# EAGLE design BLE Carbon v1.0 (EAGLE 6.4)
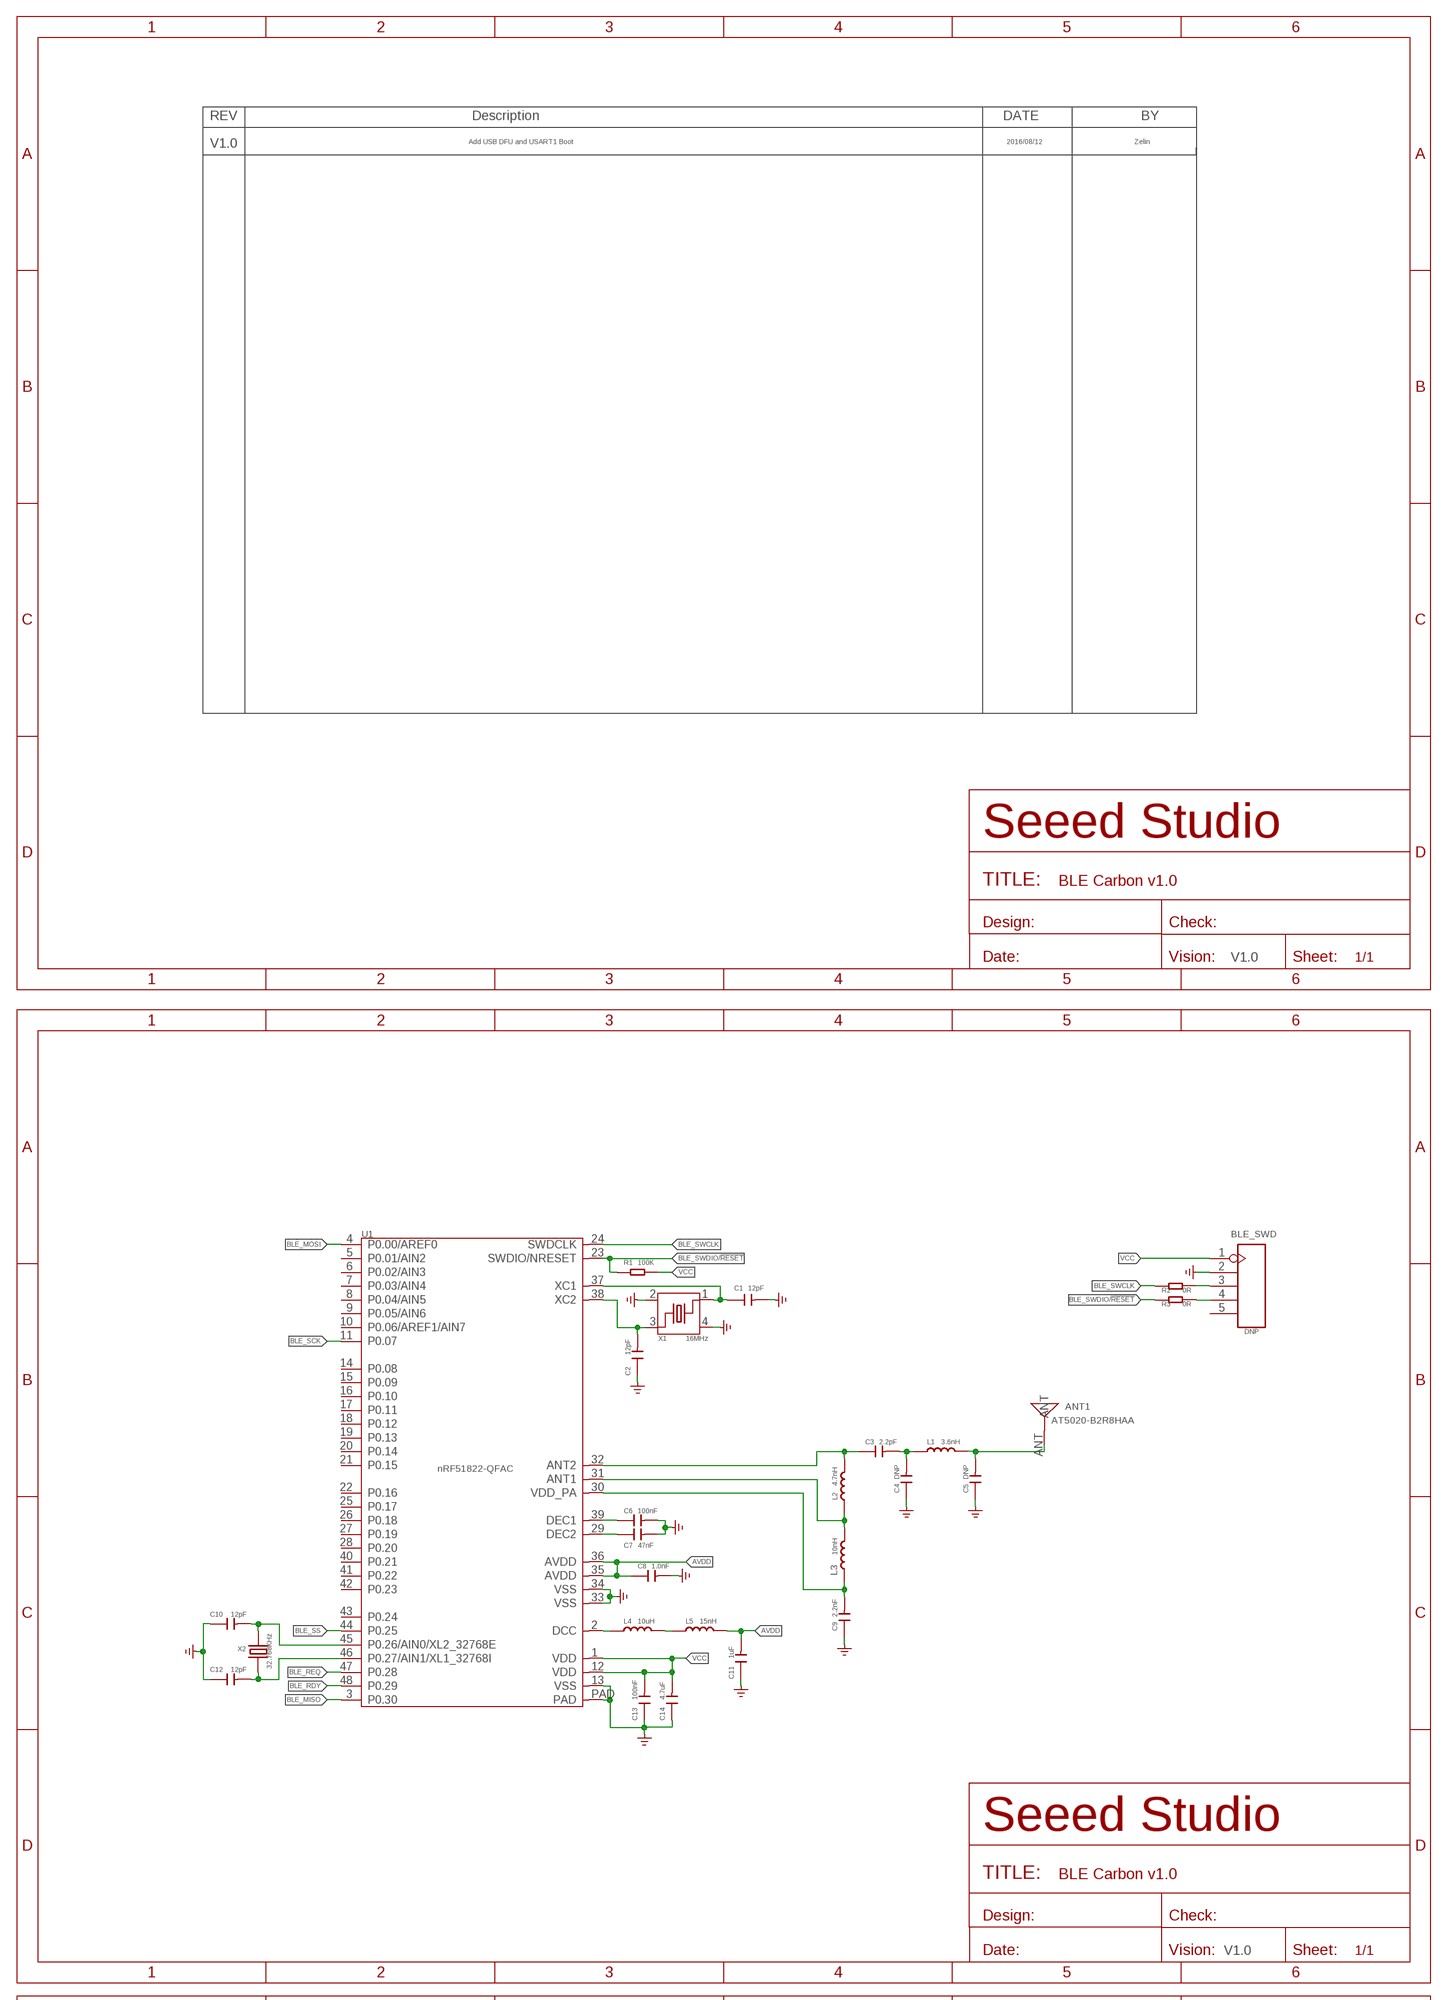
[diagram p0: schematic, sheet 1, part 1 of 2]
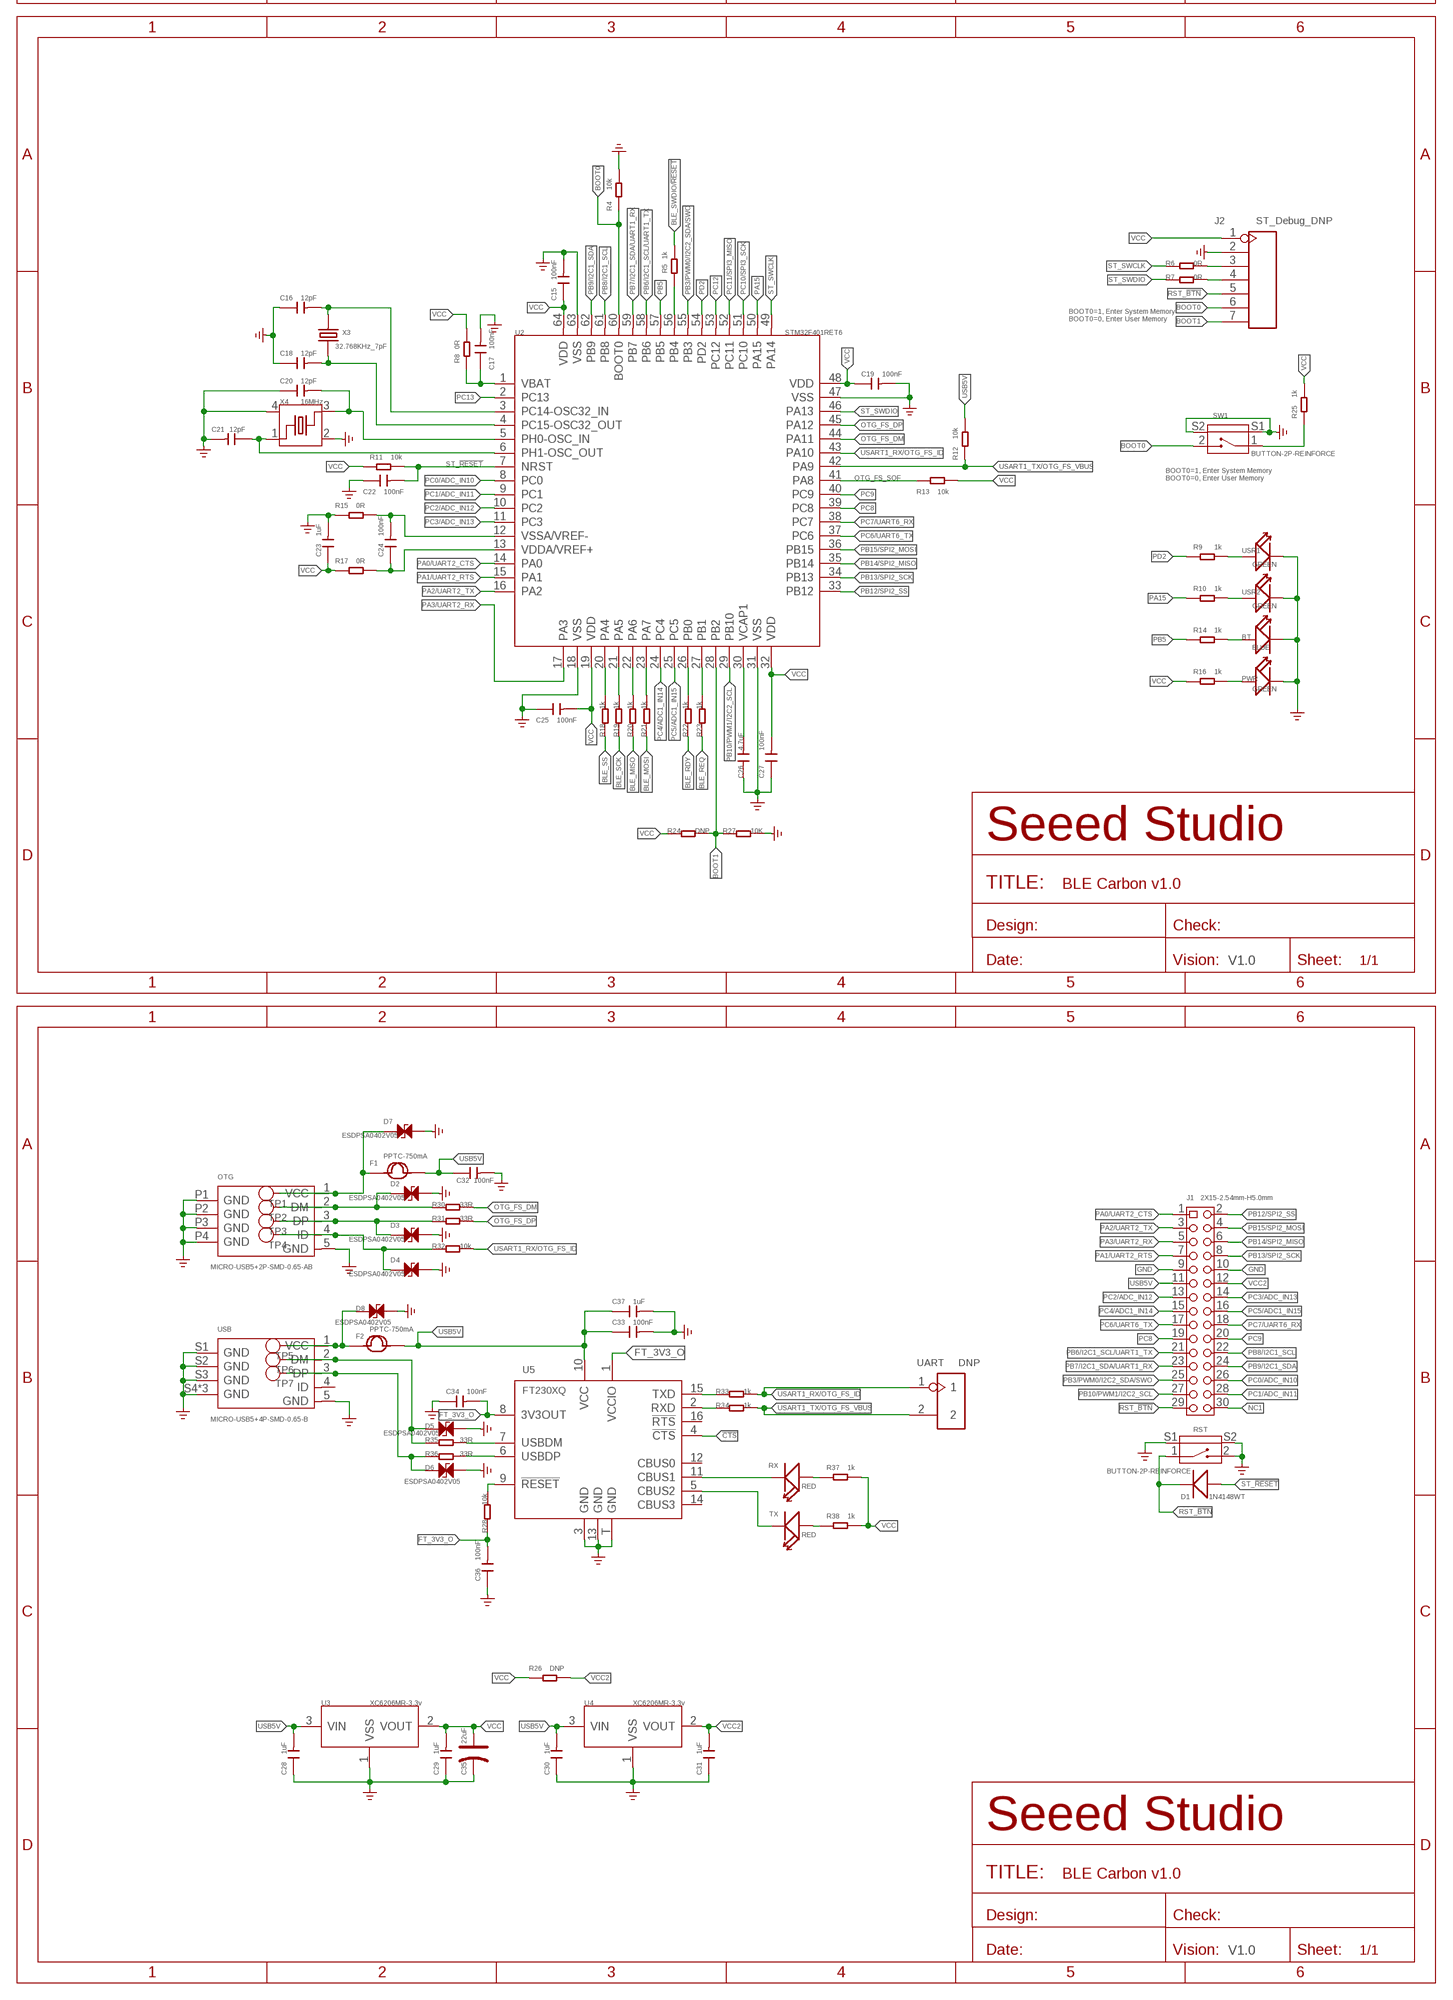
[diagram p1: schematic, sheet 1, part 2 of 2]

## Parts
ANT1  AT5020-B2R8HAA  ANTENNA-AN2051-2.4G  [ANT-SMD2P-5.05X2X1.07MM]
BLE_SWD  DNP  HEADER-5P-2.54  [H5-2.54]
BT  BLUE  LED'0402'  [LED-0402]
C1  12pF  C-0402  [C0402]
C2  12pF  C-0402  [C0402]
C3  2.2pF  C-0402  [C0402]
C4  DNP  C-0402  [C0402]
C5  DNP  C-0402  [C0402]
C6  100nF  C-0402  [C0402]
C7  47nF  C-0402  [C0402]
C8  1.0nF  C-0402  [C0402]
C9  2.2nF  C-0402  [C0402]
C10  12pF  C-0402  [C0402]
C11  1uF  C-0402  [C0402]
C12  12pF  C-0402  [C0402]
C13  100nF  C-0402  [C0402]
C14  4.7uF  C-0603  [C0603]
C15  100nF  C-0402  [C0402]
C16  12pF  C-0402  [C0402]
C17  100nF  C-0402  [C0402]
C18  12pF  C-0402  [C0402]
C19  100nF  C-0402  [C0402]
C20  12pF  C-0402  [C0402]
C21  12pF  C-0402  [C0402]
C22  100nF  C-0402  [C0402]
C23  1uF  C-0402  [C0402]
C24  100nF  C-0402  [C0402]
C25  100nF  C-0402  [C0402]
C26  4.7uF  C-0603  [C0603]
C27  100nF  C-0402  [C0402]
C28  1uF  C-0603  [C0603]
C29  1uF  C-0603  [C0603]
C30  1uF  C-0603  [C0603]
C31  1uF  C-0603  [C0603]
C32  100nF  C-0402  [C0402]
C33  100nF  C-0402  [C0402]
C34  100nF  C-0402  [C0402]
C35  22uF  CAP-AVX-A  [AVX-A]
C36  100nF  C-0402  [C0402]
C37  1uF  C-0603  [C0603]
D1  1N4148WT  D'0603'  [SOD523]
D2  ESDPSA0402V05  D-ESD-2P-DOUBLE  [ESD-0402]
D3  ESDPSA0402V05  D-ESD-2P-DOUBLE  [ESD-0402]
D4  ESDPSA0402V05  D-ESD-2P-DOUBLE  [ESD-0402]
D5  ESDPSA0402V05  D-ESD-2P-DOUBLE  [ESD-0402]
D6  ESDPSA0402V05  D-ESD-2P-DOUBLE  [ESD-0402]
D7  ESDPSA0402V05  D-ESD-2P-DOUBLE  [ESD-0402]
D8  ESDPSA0402V05  D-ESD-2P-DOUBLE  [ESD-0402]
F1  PPTC-750mA  FUSE'1206'  [F1206]
F2  PPTC-750mA  FUSE'1206'  [F1206]
J1  2X15-2.54mm-H5.0mm  HEADER-2X15P-2.54  [H2X15-2.54]
J2  ST_Debug_DNP  HEADER-7P  [H7-2.54]
L1  3.6nH  L'0402'  [L0402]
L2  4.7nH  L'0402'  [L0402]
L3  10nH  L'0402'  [L0402]
L4  10uH  L'0603'  [L0603]
L5  15nH  L'0402'  [L0402]
OTG  MICRO-USB5+2P-SMD-0.65-AB  MICRO-USB5+4P'ALX-MC-5F-036'  [MICRO-USB5+2P-SMD-0.65-AB]
PWR  GREEN  LED'0402'  [LED-0402]
R1  100K  R-0402  [R0402]
R2  0R  R-0402  [R0402]
R3  0R  R-0402  [R0402]
R4  10k  R-0402  [R0402]
R5  1k  R-0402  [R0402]
R6  0R  R-0402  [R0402]
R7  0R  R-0402  [R0402]
R8  0R  R-0402  [R0402]
R9  1k  R-0402  [R0402]
R10  1k  R-0402  [R0402]
R11  10k  R-0402  [R0402]
R12  10k  R-0402  [R0402]
R13  10k  R-0402  [R0402]
R14  1k  R-0402  [R0402]
R15  0R  R-0402  [R0402]
R16  1k  R-0402  [R0402]
R17  0R  R-0402  [R0402]
R18  1k  R-0402  [R0402]
R19  1k  R-0402  [R0402]
R20  1k  R-0402  [R0402]
R21  1k  R-0402  [R0402]
R22  1k  R-0402  [R0402]
R23  1k  R-0402  [R0402]
R24  DNP  R-0402  [R0402]
R25  1k  R-0402  [R0402]
R26  DNP  R-0402  [R0402]
R27  10K  R-0402  [R0402]
R28  10k  R-0402  [R0402]
R30  33R  R-0402  [R0402]
R31  33R  R-0402  [R0402]
R32  10k  R-0402  [R0402]
R33  1k  R-0402  [R0402]
R34  1k  R-0402  [R0402]
R35  33R  R-0402  [R0402]
R36  33R  R-0402  [R0402]
R37  1k  R-0402  [R0402]
R38  1k  R-0402  [R0402]
RST  BUTTON-2P-REINFORCE  [4P-SMD-4.7X3.5X1.8]
RX  RED  LED'0402'  [LED-0402]
SW1  BUTTON-2P-REINFORCE  [4P-SMD-4.7X3.5X1.8]
TP1  VBUS  TEST-POINT'4545'  [TP-D45MIL]
TP2  DM  TEST-POINT'4545'  [TP-D45MIL]
TP3  DP  TEST-POINT'4545'  [TP-D45MIL]
TP4  ID  TEST-POINT'4545'  [TP-D45MIL]
TP5  VBUS  TEST-POINT'4545'  [TP-D45MIL]
TP6  DM  TEST-POINT'4545'  [TP-D45MIL]
TP7  DP  TEST-POINT'4545'  [TP-D45MIL]
TX  RED  LED'0402'  [LED-0402]
U1  nRF51822-QFAC  NRF51822QFAA  [QFN48-6X6MM]
U2  STM32F401RET6  MCU-STM32F401XD/XE  [LQFP64-0.5-10X10MM]
U3  XC6206MR-3.3v  XC6206MR  [SOT23]
U4  XC6206MR-3.3v  XC6206MR  [SOT23]
U5  FT230XQ  FT230X  [QFN16]
UART  DNP  HEADER-2P-65/35MIL  [H2-2.54]
USB  MICRO-USB5+4P-SMD-0.65-B  MICRO-USB5+4P'5+4P'  [MICRO-USB5+4P-SMD-0.65-B]
USR1  GREEN  LED'0402'  [LED-0402]
USR2  GREEN  LED'0402'  [LED-0402]
X1  16MHz  CRYSTAL-4P  [X4-SMD-3.2X2.5X0.7MM]
X2  32.768KHz  CRYSTAL-3215  [2P-SMD-3.2X1.5]
X3  32.768KHz_7pF  CRYSTAL-3215  [2P-SMD-3.2X1.5]
X4  16MHz  CRYSTAL-4P  [X4-SMD-3.2X2.5X0.7MM]

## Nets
!CTS: U5.4(!CTS)
ANT1: L2.1 L3.2 U1.31(ANT1)
ANT2: C3.1 L2.2 U1.32(ANT2)
AVDD: C8.1 C11.2 L5.2 U1.35(AVDD) U1.36(AVDD)
BLE_MISO: R20.1 U1.3(P0.30)
BLE_MOSI: R21.1 U1.4(P0.00/AREF0)
BLE_RDY: R22.1 U1.48(P0.29)
BLE_REQ: R23.1 U1.47(P0.28)
BLE_SCK: R19.1 U1.11(P0.07)
BLE_SS: R18.1 U1.44(P0.25)
BLE_SWCLK: R2.1 U1.24(SWDCLK)
BLE_SWDIO/!RESET: R1.1 R3.1 R5.2 U1.23(SWDIO/NRESET)
BOOT0: J2.6 R4.1 SW1.2 U2.60(BOOT0)
BOOT1: J2.7 R24.2 R27.1 U2.28(PB2)
FT_3V3_O: C34.2 C36.2 R28.1 U5.1(VCCIO) U5.8(3V3OUT)
GND: BLE_SWD.2 BT.- C1.2 C2.1 C4.1 C5.1 C6.2 C7.2 C8.2 C9.1 C10.1 C11.1 C12.1 C13.1 C14.1 C15.2 C16.1 C17.2 C18.1 C19.2 C20.1 C21.2 C22.1 C23.2 C25.1 C26.1 C27.1 C28.1 C29.1 C30.1 C31.1 C32.2 C33.2 C34.1 C35.- C36.1 C37.2 D2.2 D3.2 D4.2 D5.2 D6.2 D7.2 D8.2 J1.9 J1.10 J2.2 OTG.5(GND) OTG.P1(GND) OTG.P2(GND) OTG.P3(GND) OTG.P4(GND) PWR.- R4.2 R15.1 R27.2 RST.2 RST.S1 RST.S2 SW1.S1 SW1.S2 U1.13(VSS) U1.33(VSS) U1.34(VSS) U1.PAD U2.18(VSS) U2.31(VSS) U2.47(VSS) U2.63(VSS) U3.1(VSS) U4.1(VSS) U5.3(GND) U5.13(GND) U5.T(GND) USB.5(GND) USB.S1(GND) USB.S2(GND) USB.S3(GND) USB.S4(GND) USB.S5(GND) USB.S6(GND) USR1.- USR2.- X1.2 X1.4 X4.2 X4.4 ; supply symbol labelled GND_POWER
N$1: ANT1.ANT C5.2 L1.2
N$2: C2.2 U1.38(XC2) X1.3
N$3: C7.1 U1.29(DEC2)
N$4: C6.1 U1.39(DEC1)
N$5: C1.1 U1.37(XC1) X1.1
N$6: L4.1 U1.2(DCC)
N$7: L4.2 L5.1
N$8: C3.2 C4.2 L1.1
N$9: C26.2 U2.30(VCAP1)
N$10: J2.3 R6.2
N$11: D4.1 OTG.4(ID) R32.1 TP4.T
N$12: C21.1 U2.6(PH1-OSC_OUT) X4.1
N$13: C20.2 U2.5(PH0-OSC_IN) X4.3
N$14: D2.1 OTG.2(DM) R30.1 TP2.T
N$15: D3.1 OTG.3(DP) R31.1 TP3.T
N$17: D8.1 F2.1 TP5.T USB.1(VCC)
N$18: C17.1 R8.1 U2.1(VBAT)
N$19: R18.2 U2.20(PA4)
N$20: R19.2 U2.21(PA5)
N$21: R20.2 U2.22(PA6)
N$22: R21.2 U2.23(PA7)
N$23: R22.2 U2.26(PB0)
N$24: R23.2 U2.27(PB1)
N$25: R25.1 SW1.1
N$26: C24.2 R15.2 U2.12(VSSA/VREF-)
N$27: C24.1 R17.2 U2.13(VDDA/VREF+)
N$28: BLE_SWD.4 R3.2
N$29: J2.4 R7.2
N$30: R35.2 U5.7(USBDM)
N$31: R9.2 USR1.+
N$32: R36.2 U5.6(USBDP)
N$33: R33.1 U5.15(TXD)
N$34: R34.1 U5.2(RXD)
N$35: R10.2 USR2.+
N$36: BT.+ R14.2
N$37: R5.1 U2.56(PB4)
N$38: R28.2 U5.9(!RESET)
N$39: D7.1 F1.1 OTG.1(VCC) TP1.T
N$40: BLE_SWD.3 R2.2
N$41: RX.- U5.11(CBUS1)
N$42: PWR.+ R16.2
N$43: TX.- U5.5(CBUS2)
N$44: R37.1 RX.+
N$45: R38.1 TX.+
N$46: D5.1 R35.1 TP6.T USB.2(DM)
N$47: D6.1 R36.1 TP7.T USB.3(DP)
NC1: J1.30
OTG_FS_DM: R30.2 U2.44(PA11)
OTG_FS_DP: R31.2 U2.45(PA12)
OTG_FS_SOF: R13.1 U2.41(PA8)
PA0/UART2_CTS: J1.1 U2.14(PA0)
PA1/UART2_RTS: J1.7 U2.15(PA1)
PA2/UART2_TX: J1.3 U2.16(PA2)
PA3/UART2_RX: J1.5 U2.17(PA3)
PA15: R10.1 U2.50(PA15)
PB3/PWM0/I2C2_SDA/SWO: J1.25 U2.55(PB3)
PB5: R14.1 U2.57(PB5)
PB6/I2C1_SCL/UART1_TX: J1.21 U2.58(PB6)
PB7/I2C1_SDA/UART1_RX: J1.23 U2.59(PB7)
PB8/I2C1_SCL: J1.22 U2.61(PB8)
PB9/I2C1_SDA: J1.24 U2.62(PB9)
PB10/PWM1/I2C2_SCL: J1.27 U2.29(PB10)
PB12/SPI2_SS: J1.2 U2.33(PB12)
PB13/SPI2_SCK: J1.8 U2.34(PB13)
PB14/SPI2_MISO: J1.6 U2.35(PB14)
PB15/SPI2_MOSI: J1.4 U2.36(PB15)
PC0/ADC_IN10: J1.26 U2.8(PC0)
PC1/ADC_IN11: J1.28 U2.9(PC1)
PC2/ADC_IN12: J1.13 U2.10(PC2)
PC3/ADC_IN13: J1.14 U2.11(PC3)
PC4/ADC1_IN14: J1.15 U2.24(PC4)
PC5/ADC1_IN15: J1.16 U2.25(PC5)
PC6/UART6_TX: J1.17 U2.37(PC6)
PC7/UART6_RX: J1.18 U2.38(PC7)
PC8: J1.19 U2.39(PC8)
PC9: J1.20 U2.40(PC9)
PC10/SPI3_SCK: U2.51(PC10)
PC11/SPI3_MISO: U2.52(PC11)
PC12: U2.53(PC12)
PC13: U2.2(PC13)
PD2: R9.1 U2.54(PD2)
RST_!BTN: D1.- J1.29 J2.5 RST.1
ST_!RESET: C22.2 D1.+ R11.2 U2.7(NRST)
ST_SWCLK: R6.1 U2.49(PA14)
ST_SWDIO: R7.1 U2.46(PA13)
USART1_RX/OTG_FS_ID: R32.2 R33.2 U2.43(PA10) UART.1
USART1_TX/OTG_FS_VBUS: R12.1 R34.2 U2.42(PA9) UART.2
USB5V: C28.2 C30.2 C32.1 C33.1 C37.1 F1.2 F2.2 J1.11 R12.2 U3.3(VIN) U4.3(VIN) U5.10(VCC)
VCC: BLE_SWD.1 C13.2 C14.2 C15.1 C19.1 C23.1 C25.2 C27.2 C29.2 C35.+ J2.1 R1.2 R8.2 R11.1 R13.2 R16.1 R17.1 R24.1 R25.2 R26.1 R37.2 R38.2 U1.1(VDD) U1.12(VDD) U2.19(VDD) U2.32(VDD) U2.48(VDD) U2.64(VDD) U3.2(VOUT)
VCC2: C31.2 J1.12 R26.2 U4.2(VOUT)
VDD_PA: C9.2 L3.1 U1.30(VDD_PA)
XL1_32768I: C12.2 U1.46(P0.27/AIN1/XL1_32768I) X2.1
XL1_32768I1: C18.2 U2.4(PC15-OSC32_OUT) X3.1
XL2_32768E: C10.2 U1.45(P0.26/AIN0/XL2_32768E) X2.2
XL2_32768E1: C16.2 U2.3(PC14-OSC32_IN) X3.2
Unconnected: BLE_SWD.5 U1.5(P0.01/AIN2) U1.6(P0.02/AIN3) U1.7(P0.03/AIN4) U1.8(P0.04/AIN5) U1.9(P0.05/AIN6) U1.10(P0.06/AREF1/AIN7) U1.14(P0.08) U1.15(P0.09) U1.16(P0.10) U1.17(P0.11) U1.18(P0.12) U1.19(P0.13) U1.20(P0.14) U1.21(P0.15) U1.22(P0.16) U1.25(P0.17) U1.26(P0.18) U1.27(P0.19) U1.28(P0.20) U1.40(P0.21) U1.41(P0.22) U1.42(P0.23) U1.43(P0.24) U5.12(CBUS0) U5.14(CBUS3) U5.16(!RTS) USB.4(ID)

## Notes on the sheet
- Add USB DFU and USART1 Boot | 2016/08/12 | Zelin
- V1.0
- V1.0
- V1.0
- BOOT0=1, Enter System Memory
  BOOT0=0, Enter User Memory
- BOOT0=1, Enter System Memory
  BOOT0=0, Enter User Memory
- V1.0
- V1.0

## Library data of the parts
ANT1 = Connector-new:ANTENNA-AN2051-2.4G: Multilayer Chip Antenna for 2.4GHz Wireless Communication
BLE_SWD = Connector-update:HEADER-5P
BT PWR RX TX USR1 USR2 = Discrete:LED*
C1-C34 C36 C37 = Discrete:C*: Ceramic Capacitors
C35 = Discrete:CAP*: Electrolytic Capacitors,Tantalum Capacitors and Super Capacitors
D1 = Discrete:D*
D2-D8 = Discrete-new:D-ESD-2P-DOUBLE
F1 F2 = Discrete:FUSE
J1 = Connector-update:HEADER-2X15P
J2 = Connector-new:HEADER-7P
L1-L5 = Discrete:L*
OTG = Connector-new:MICRO-USB5+4P: 5+4P-SMD-0.65-B:320010000;5+2P-SMD-0.65-AB:340032001; MPN: ALX-MC-5F-036; SKU: 320010025
R1-R28 R30-R38 = Discrete:R*
RST SW1 = Discrete:BUTTON-2P-REINFORCE: TS-1188E http://www.best-dz.com/?thread-374-2.html SMD Button
TP1-TP7 = Discrete-new:TEST-POINT; PARTNO: DNP
U1 = AMLib_New:NRF51822QFAA: Multi-protocol Blutooth 4.0 low energy /2. GHz RF SoC
U2 = AMLib_U2N:MCU-STM32F401XD/XE
U3 U4 = IC:XC6206: LOW ESR Cap.Compatible Positive Voltage Regulators
U5 = AMLib_New:FT230X
UART = Connector-update:HEADER-2P
USB = Connector-new:MICRO-USB5+4P: 5+4P-SMD-0.65-B:320010000;5+2P-SMD-0.65-AB:340032001
X1 X4 = Discrete-new:CRYSTAL-4P
X2 X3 = Discrete:CRYSTAL*: CRYSTAL

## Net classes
0 default: width 0.152 mm, drill 0.254 mm, clearance 0.152 mm
1 vcc: width 0.203 mm

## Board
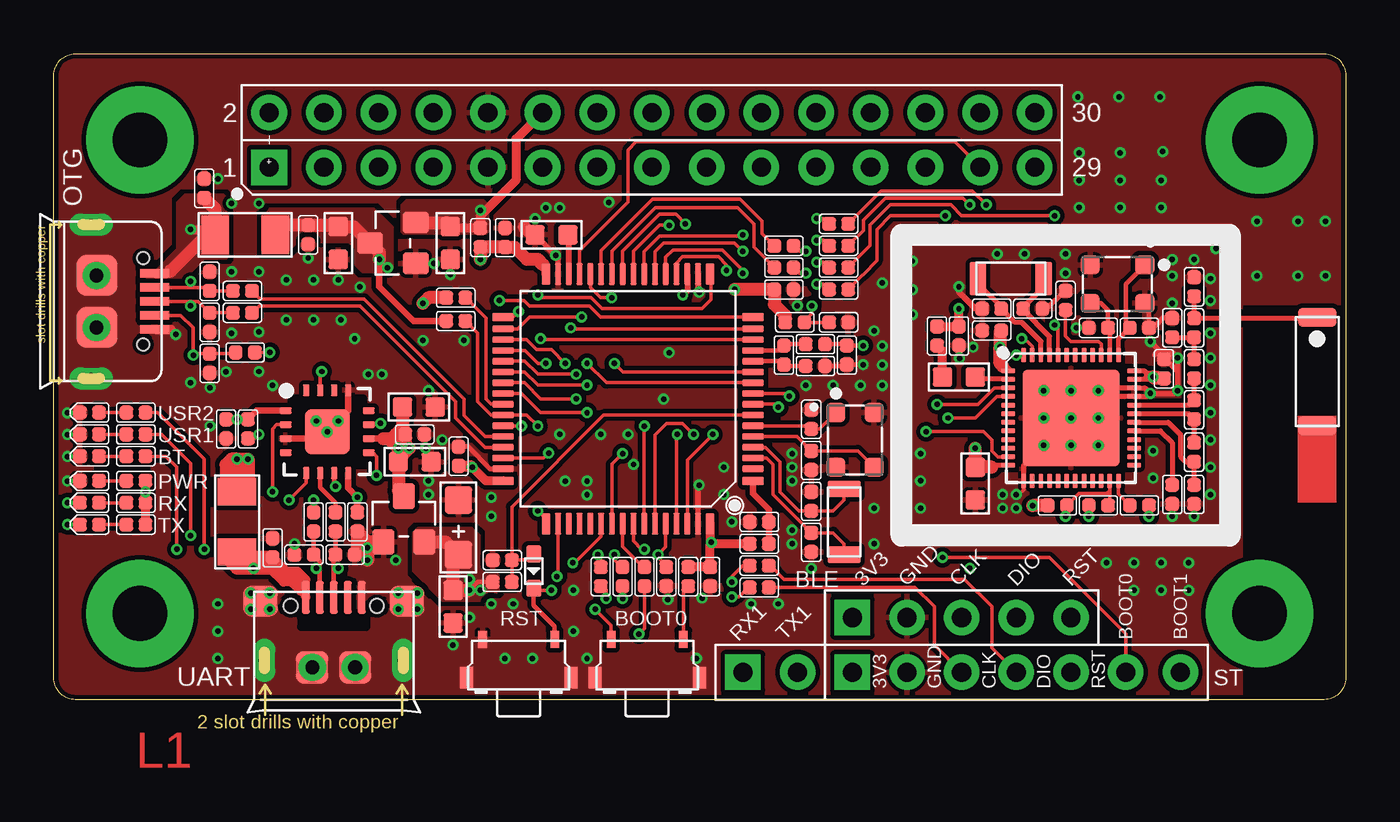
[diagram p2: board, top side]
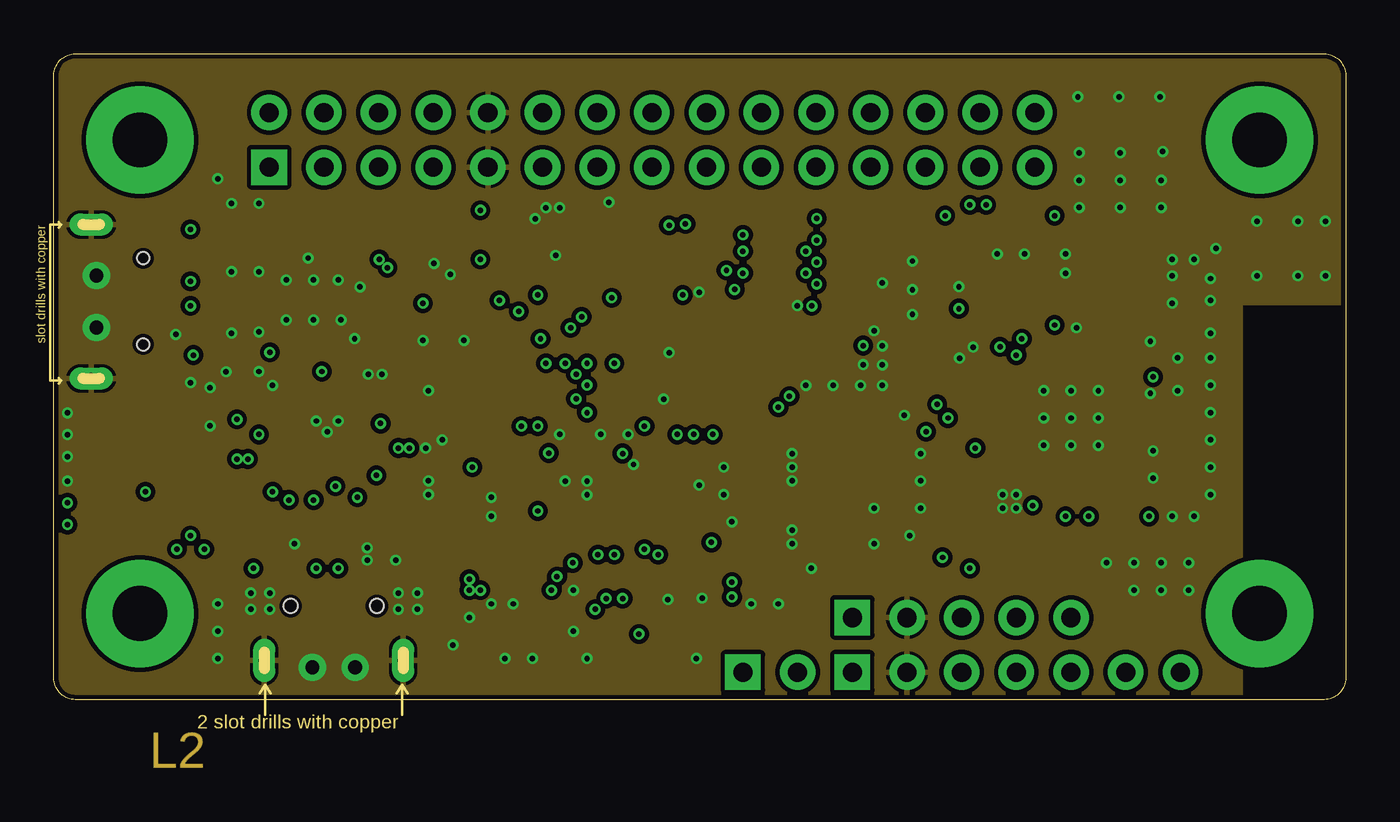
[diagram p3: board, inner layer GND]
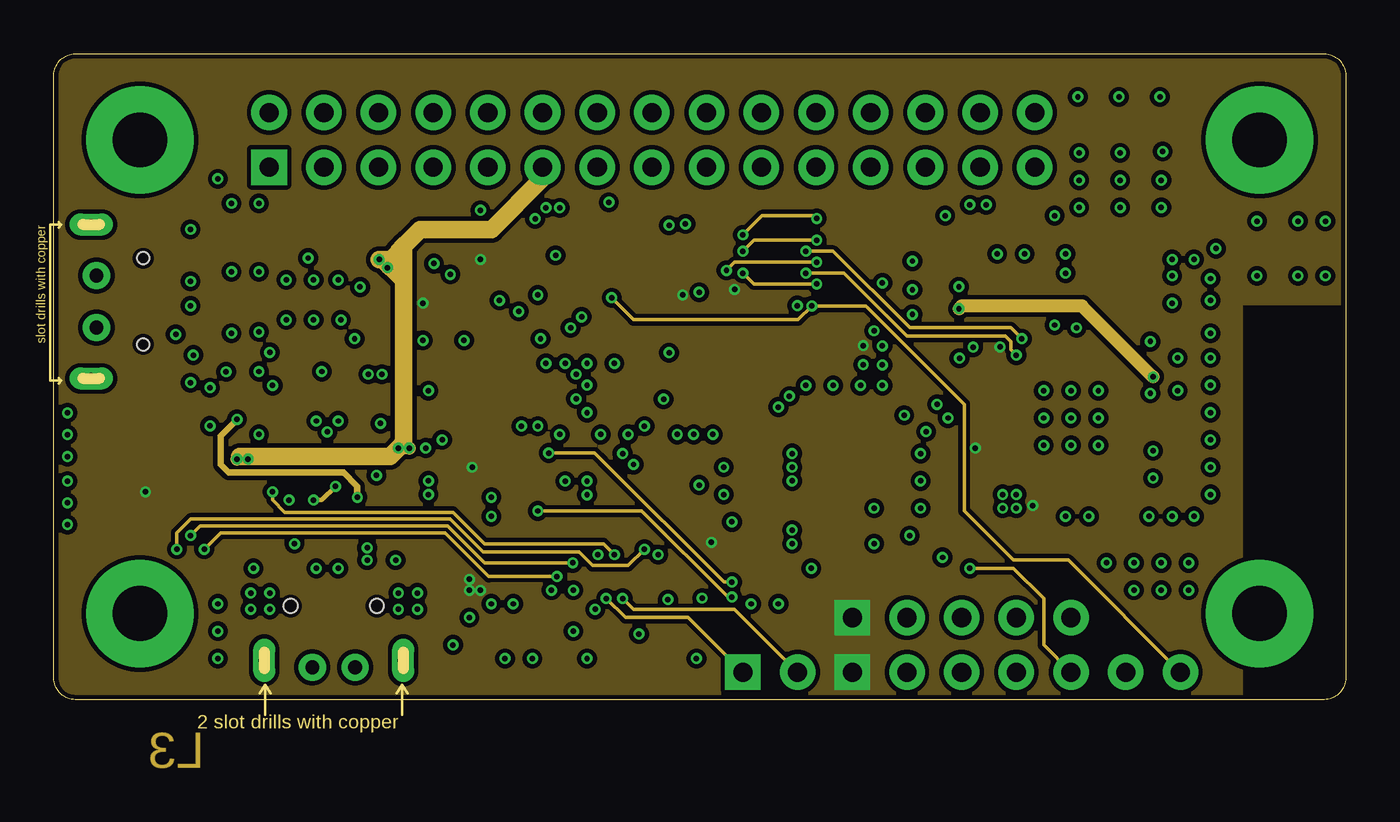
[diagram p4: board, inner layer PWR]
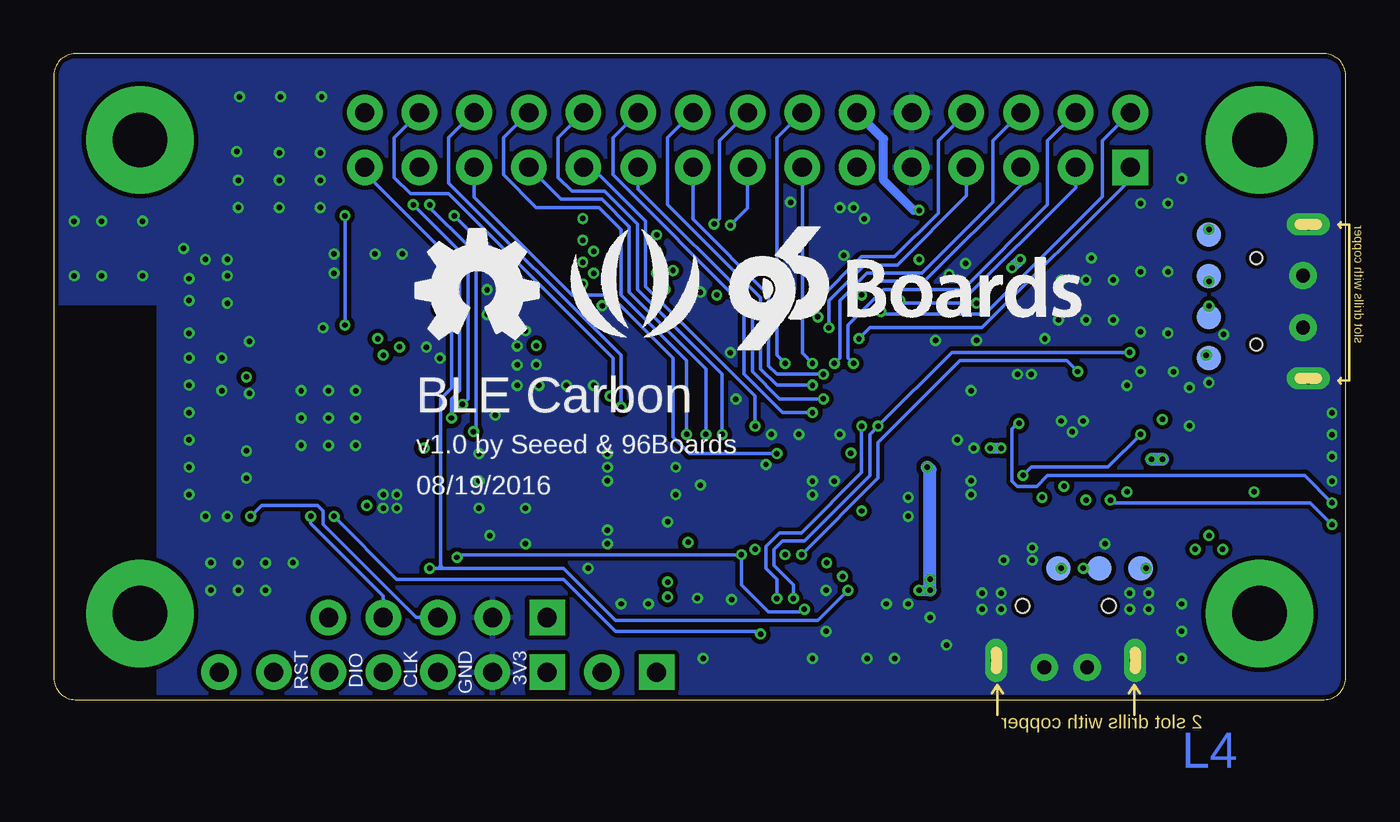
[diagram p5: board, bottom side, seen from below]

Size 60 x 30 mm. Coordinates in mm from the lower left corner, seen from the top.
Outline: 1,30 59,30 arc-90 60,29 60,1 arc-90 59,0 1,0 arc-90 0,1 0,29 arc-90 1,30
Copper layers (1*2*15*16): Top 0.035mm / dielectric 0.2mm / GND 0.0175mm / dielectric 0.3mm / PWR 0.0175mm / dielectric 0.2mm / Bottom 0.035mm
Design rules "SeeedStudio_4layer_DRU_no_angle_20140221 *": minimum track width 1mil, minimum drill 10mil, track to track 6mil, track to pad 6mil, pad to pad 6mil, via to via 6mil, smd to smd 0mil, copper to edge 8mil, drill to drill 8mil, minimum pad ring 4mil, minimum via ring 4mil, stop-mask expansion 4mil, vias tented up to drill 20mil, thermal gap 6mil
tRestrict: area 11,10.9 to 14.4,14; area 57.3,12.4 to 60.1,18; area 52.6,9.7 to 53.3,19.1; area 53.3,17.5 to 55.2,17.9
bRestrict: area 57.3,12.4 to 60.1,18

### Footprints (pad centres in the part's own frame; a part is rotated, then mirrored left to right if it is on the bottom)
ANT-SMD2P-5.05X2X1.07MM = smd 1.8 x 0.9: ANT 0,2.513; P$1 0,-2.513
H5-2.54 = drill 0.889 pad 1.651 square: 1 0,5.08 | drill 0.889 pad 1.651: 2 0,2.54; 3 0,0; 4 0,-2.54; 5 0,-5.08
LED-0402 = smd 0.635 x 0.635: + -0.445,0; - 0.445,0
C0402 = smd 0.635 x 0.635: 1 -0.445,0; 2 0.445,0
C0603 = smd 0.889 x 0.889: 1 -0.762,0; 2 0.762,0
AVX-A = smd 1.27 x 1.27: + -1.27,0; - 1.27,0
SOD523 = smd 0.762 x 0.7: + -0.8,0; - 0.8,0
ESD-0402 = smd 0.635 x 0.635: 1 -0.445,0; 2 0.445,0
F1206 = smd 1.27 x 1.778: 1 -1.397,0; 2 1.397,0
H2X15-2.54 = drill 0.889 pad 1.651 square: 1 -1.27,0 | drill 0.889 pad 1.651: 2 1.27,0; 3 -1.27,-2.54; 4 1.27,-2.54; 5 -1.27,-5.08; 6 1.27,-5.08; 7 -1.27,-7.62; 8 1.27,-7.62; 9 -1.27,-10.16; 10 1.27,-10.16; 11 -1.27,-12.7; 12 1.27,-12.7; 13 -1.27,-15.24; 14 1.27,-15.24; 15 -1.27,-17.78; 16 1.27,-17.78; 17 -1.27,-20.32; 18 1.27,-20.32; 19 -1.27,-22.86; 20 1.27,-22.86; 21 -1.27,-25.4; 22 1.27,-25.4; 23 -1.27,-27.94; 24 1.27,-27.94; 25 -1.27,-30.48; 26 1.27,-30.48; 27 -1.27,-33.02; 28 1.27,-33.02; 29 -1.27,-35.56; 30 1.27,-35.56
H7-2.54 = drill 0.889 pad 1.651 square: 1 0,7.62 | drill 0.889 pad 1.651: 2 0,5.08; 3 0,2.54; 4 0,0; 5 0,-2.54; 6 0,-5.08; 7 0,-7.62
L0402 = smd 0.635 x 0.635: 1 -0.445,0; 2 0.445,0
L0603 = smd 0.889 x 0.889: 1 -0.762,0; 2 0.762,0
MICRO-USB5+2P-SMD-0.65-AB = smd 0.4 x 1.35: 1 -1.3,2.675; 2 -0.65,2.675; 3 0,2.675; 4 0.65,2.675; 5 1.3,2.675 | smd 1.9 x 1.9: P1 -1.2,0; P2 1.2,0 | drill 0.508 pad 1.016 long: P3 -3.575,-0.265; P4 3.575,-0.265 | hole 0.55: -2,2.15; 2,2.15
R0402 = smd 0.635 x 0.635: 1 -0.445,0; 2 0.445,0
4P-SMD-4.7X3.5X1.8 = smd 0.4 x 0.8: 1 -1.675,-1.277; 2 1.675,-1.277 | smd 0.6 x 1: S1 -2.425,0.5; S2 2.425,0.5
TP-D45MIL = smd 1.143 x 1.143: T 0,0
QFN48-6X6MM = smd 0.23 x 0.65: 1 -2.2,-2.925; 2 -1.8,-2.925; 3 -1.4,-2.925; 4 -1,-2.925; 5 -0.6,-2.925; 6 -0.2,-2.925; 7 0.2,-2.925; 8 0.6,-2.925; 9 1,-2.925; 10 1.4,-2.925; 11 1.8,-2.925; 12 2.2,-2.925; 25 2.2,2.925; 26 1.8,2.925; 27 1.4,2.925; 28 1,2.925; 29 0.6,2.925; 30 0.2,2.925; 31 -0.2,2.925; 32 -0.6,2.925; 33 -1,2.925; 34 -1.4,2.925; 35 -1.8,2.925; 36 -2.2,2.925 | smd 0.65 x 0.23: 13 2.925,-2.2; 14 2.925,-1.8; 15 2.925,-1.4; 16 2.925,-1; 17 2.925,-0.6; 18 2.925,-0.2; 19 2.925,0.2; 20 2.925,0.6; 21 2.925,1; 22 2.925,1.4; 23 2.925,1.8; 24 2.925,2.2; 37 -2.925,2.2; 38 -2.925,1.8; 39 -2.925,1.4; 40 -2.925,1; 41 -2.925,0.6; 42 -2.925,0.2; 43 -2.925,-0.2; 44 -2.925,-0.6; 45 -2.925,-1; 46 -2.925,-1.4; 47 -2.925,-1.8; 48 -2.925,-2.2 | smd 4.5 x 4.5: PAD 0,0
LQFP64-0.5-10X10MM = smd 1 x 0.4: 1 -5.8,3.81; 16 -5.8,-3.81; 33 5.8,-3.81; 48 5.8,3.81 | smd 1 x 0.28: 2 -5.8,3.25; 3 -5.8,2.75; 4 -5.8,2.25; 5 -5.8,1.75; 6 -5.8,1.25; 7 -5.8,0.75; 8 -5.8,0.25; 9 -5.8,-0.25; 10 -5.8,-0.75; 11 -5.8,-1.25; 12 -5.8,-1.75; 13 -5.8,-2.25; 14 -5.8,-2.75; 15 -5.8,-3.25; 34 5.8,-3.25; 35 5.8,-2.75; 36 5.8,-2.25; 37 5.8,-1.75; 38 5.8,-1.25; 39 5.8,-0.75; 40 5.8,-0.25; 41 5.8,0.25; 42 5.8,0.75; 43 5.8,1.25; 44 5.8,1.75; 45 5.8,2.25; 46 5.8,2.75; 47 5.8,3.25 | smd 0.4 x 1: 17 -3.81,-5.8; 32 3.81,-5.8; 49 3.81,5.8; 64 -3.81,5.8 | smd 0.28 x 1: 18 -3.25,-5.8; 19 -2.75,-5.8; 20 -2.25,-5.8; 21 -1.75,-5.8; 22 -1.25,-5.8; 23 -0.75,-5.8; 24 -0.25,-5.8; 25 0.25,-5.8; 26 0.75,-5.8; 27 1.25,-5.8; 28 1.75,-5.8; 29 2.25,-5.8; 30 2.75,-5.8; 31 3.25,-5.8; 50 3.25,5.8; 51 2.75,5.8; 52 2.25,5.8; 53 1.75,5.8; 54 1.25,5.8; 55 0.75,5.8; 56 0.25,5.8; 57 -0.25,5.8; 58 -0.75,5.8; 59 -1.25,5.8; 60 -1.75,5.8; 61 -2.25,5.8; 62 -2.75,5.8; 63 -3.25,5.8
SOT23 = smd 1.016 x 1.2: 1 -0.95,-1.06; 2 0.95,-1.06; 3 0,1.06
QFN16 = smd 0.55 x 0.3: 1 -1.925,0.975; 2 -1.925,0.325; 3 -1.925,-0.325; 4 -1.925,-0.975; 9 1.925,-0.975; 10 1.925,-0.325; 11 1.925,0.325; 12 1.925,0.975 | smd 0.3 x 0.55: 5 -0.975,-1.925; 6 -0.325,-1.925; 7 0.325,-1.925; 8 0.975,-1.925; 13 0.975,1.925; 14 0.325,1.925; 15 -0.325,1.925; 16 -0.975,1.925 | smd 2.1 x 2.1: T 0,0
96BOARDS_IOT_EDITION_STANDARD = drill 2.54 pad 5: P$1 4,26; P$2 4,4; P$3 56,4; P$4 56,26
H2-2.54 = drill 0.889 pad 1.651 square: 1 0,1.27 | drill 0.889 pad 1.651: 2 0,-1.27
MICRO-USB5+4P-SMD-0.65-B = smd 0.381 x 1.524: 1 -1.3,-0.25; 2 -0.65,-0.25; 3 0,-0.25; 4 0.65,-0.25; 5 1.3,-0.25 | smd 1.6 x 1.397: S1 -3.4,-0.427; S6 3.4,-0.427 | drill 0.508 pad 1.016 long: S2 -3.226,-3.175; S5 3.226,-3.175 | smd 1.5 x 1.5: S3 -1,-3.5; S4 1,-3.5 | hole 0.635: -2,-0.65; 2,-0.65
X4-SMD-3.2X2.5X0.7MM = smd 0.889 x 0.889: 1 -1.27,-0.889; 2 1.27,-0.889; 3 1.27,0.889; 4 -1.27,0.889
2P-SMD-3.2X1.5 = smd 0.762 x 1.524: 1 -1.524,0; 2 1.524,0

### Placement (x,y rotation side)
ANT1  58.67,15.24 0 top
BLE_SWD  42.16,3.81 90 top
BT  1.65,11.3 180 top
C1  50.42,17.27 0 top
C2  48.51,17.27 0 top
C3  52.96,15.37 90 top
C4  51.94,17.27 270 top
C5  52.96,19.18 270 top
C6  46.99,18.54 90 top
C7  51.94,9.53 270 top
C8  51.56,15.37 90 top
C9  52.96,9.53 90 top
C10  45.47,18.16 180 top
C11  42.04,16.89 90 top
C12  43.56,18.16 0 top
C13  43.56,17.14 0 top
C14  42.8,10.03 90 top
C15  30.48,5.71 270 top
C16  35.18,7.3 90 top
C17  32.77,8.26 180 top
C18  35.18,9.21 270 top
C19  18.8,11.3 90 top
C20  35.18,11.11 90 top
C21  35.18,13.02 90 top
C22  20.83,6.48 0 top
C23  36.83,16 270 top
C24  33.91,16 270 top
C25  33.91,19.05 180 top
C26  23.11,21.59 0 top
C27  20.95,21.46 270 top
C28  16.76,11.05 180 top
C29  18.54,4.32 90 top
C30  13.21,21.21 90 top
C31  18.41,21.21 90 top
C32  11.81,21.59 270 top
C33  16.76,12.32 0 top
C34  14.1,8.26 90 top
C35  18.8,8 90 top
C36  8,12.57 90 top
C37  16.95,13.59 0 top
D1  22.29,5.97 270 top
D2  7.24,19.43 90 top
D3  7.24,17.53 270 top
D4  7.24,15.62 270 top
D5  11.62,6.73 180 top
D6  13.53,6.73 0 top
D7  6.99,23.75 90 top
D8  10.16,7.05 90 top
F1  8.89,21.59 0 top
F2  8.51,8.26 90 top
J1  10,26 90 top
J2  44.7,1.27 90 top
L1  52.96,17.27 90 top
L2  52.96,13.46 90 top
L3  52.96,11.49 90 top
L4  42.04,14.99 180 top
L5  41.02,16.89 90 top
OTG  2,18.5 270 top
PWR  1.65,10.16 180 top
R1  46.61,9.02 180 top
R2  50.42,9.02 0 top
R3  48.51,9.02 180 top
R4  28.45,5.71 270 top
R5  27.43,5.71 270 top
R6  32.77,5.21 0 top
R7  32.77,6.22 0 top
R8  32.77,7.24 180 top
R9  3.81,12.32 180 top
R10  3.81,13.34 180 top
R11  20.83,5.46 0 top
R12  18.67,17.59 180 top
R13  18.67,18.67 180 top
R14  3.81,11.3 180 top
R15  35.37,15.49 180 top
R16  3.81,10.16 180 top
R17  35.37,16.51 180 top
R18  36.45,20.07 180 top
R19  36.45,19.05 180 top
R20  36.45,21.08 180 top
R21  36.45,22.1 180 top
R22  33.91,20.07 180 top
R23  33.91,21.08 180 top
R24  34.42,17.53 0 top
R25  29.46,5.71 90 top
R26  19.81,21.46 90 top
R27  36.45,17.53 0 top
R28  9.02,12.57 270 top
R30  8.76,18.99 0 top
R31  8.76,17.97 0 top
R32  8.89,16.13 0 top
R33  25.4,5.71 270 top
R34  26.42,5.71 270 top
R35  12.06,8.26 90 top
R36  13.08,8.26 90 top
R37  3.81,9.14 0 top
R38  3.81,8.13 0 top
RST  21.59,1.52 180 top
RX  1.65,9.14 180 top
SW1  27.56,1.52 180 top
TP1  6.35,21.59 0 bottom
TP2  6.35,19.68 0 bottom
TP3  6.35,17.78 0 bottom
TP4  6.35,15.88 0 bottom
TP5  9.53,6.1 270 bottom
TP6  11.43,6.1 270 bottom
TP7  13.34,6.1 270 bottom
TX  1.65,8.13 180 top
U1  47.24,13.08 270 top
U2  26.67,13.97 180 top
U3  16.26,8.38 0 top
U4  15.75,21.21 90 top
U5  12.7,12.45 0 top
U$8  [96BOARDS_IOT_EDITION_STANDARD]  0,0 0 top
U$48  [SEEED-SILK-280*268MIL]  33.01,18.54 0 bottom
U$49  [96BOARDS_SILK]  28.95,15.75 0 bottom
U$50  [OSHW_FILLX200_NOTEXT]  43.17,16.76 0 bottom
UART  33.27,1.27 90 top
USB  13,5 0 top
USR1  1.65,12.32 180 top
USR2  1.65,13.34 180 top
X1  49.4,19.3 180 top
X2  44.45,19.56 0 top
X3  36.7,8.26 270 top
X4  37.21,12.06 270 top

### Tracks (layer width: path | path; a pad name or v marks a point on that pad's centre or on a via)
ANT1
  Top 0.229: U1.31 52.7,13.28 L2.1 L3.2
ANT2
  Top 0.229: U1.32 52.73,13.68 L2.2 C3.1
AVDD  (via drill 0.25 pad 0.51)
  Top 0.229: U1.35 50.91,14.88 50.93,14.86 50.93,14.99 | U1.36 50.63,15.28 50.75,15.16 | 50.75,15.16 50.93,14.99 | 50.93,14.99 v51.05,14.99 | 50.75,15.16 50.75,14.99 50.67,14.91 | 50.75,15.16 51.28,15.16 51.49,14.96
  Top 0.406: L5.2 C11.2 v42.04,18.16
  Top 0.61: C8.1 51.12,14.92 v51.05,14.99
  PWR 0.61: v51.05,14.99 47.75,18.29 42.16,18.29 v42.04,18.16
BLE_MISO  (via drill 0.25 pad 0.51)
  Top 0.152: U1.3 43.69,14.48 42.93,13.72 v41.02,13.72 | R20.1 37.59,21.78 37.59,22.26 38.63,23.3 42.23,23.3 v42.55,22.99
  Bottom 0.152: v42.55,22.99 42.55,22.86 40.77,21.08 40.77,13.97 v41.02,13.72
BLE_MOSI  (via drill 0.25 pad 0.51)
  Top 0.152: U1.4 43.8,14.08 42.8,13.08 v41.53,13.08 | v43.31,22.99 42.67,23.62 38.42,23.62 R21.1
  Bottom 0.152: v43.31,22.99 41.15,20.83 41.15,14.35 41.53,13.97 v41.53,13.08
BLE_RDY  (via drill 0.25 pad 0.51)
  Top 0.152: U1.48 v44.71,16.01 v44.7,16 | v34.92,19.81 34.61,19.81 R22.1
  PWR 0.152: v44.7,16 44.45,16.26 44.45,16.64 44.2,16.89 39.62,16.89 36.7,19.81 v34.92,19.81
BLE_REQ  (via drill 0.25 pad 0.51)
  Top 0.152: U1.47 45.44,16.41 45.09,16.76 v44.96,16.76 | v34.92,20.83 34.61,20.83 R23.1
  PWR 0.152: v44.96,16.76 44.45,17.27 39.75,17.27 36.2,20.83 v34.92,20.83
BLE_SCK  (via drill 0.25 pad 0.51)
  Top 0.152: U1.11 43.84,11.28 43.56,11.56 43.56,12.06 43.18,12.45 v40.51,12.45 | R19.1 37.56,19.72 37.59,19.75 38.23,20.38 38.23,21.84 38.86,22.48 v41.4,22.48
  Bottom 0.152: v41.4,22.48 40.39,21.46 40.39,12.57 v40.51,12.45
BLE_SS  (via drill 0.25 pad 0.51)
  Top 0.152: U1.44 46.64,17.24 v46.48,17.4 | 36.89,20.13 R18.1 37.91,21.08 37.91,22.04 38.86,22.99 41.66,22.99 42.16,22.48 v46.48,22.48
  Bottom 0.152: v46.48,22.48 v46.48,17.4
BLE_SWCLK
  Top 0.152: U1.24 49.44,9.55 R2.1
BLE_SWDIO/!RESET  (via drill 0.25 pad 0.51)
  Top 0.152: 48.9,9.58 48.99,9.58 49.04,9.53 | 48.9,9.58 47.61,9.58 R1.1 47.05,8.57 v46.99,8.51 | U1.23 49.04,9.53 | 49.04,9.53 49.04,9.1 R3.1 | 48.9,9.58 49.02,9.45 | 48.9,9.58 49.02,9.7 | R5.2 27.43,3.3 v27.18,3.05
  Bottom 0.152: v27.18,3.05 27.3,3.17 33.91,3.17 36.32,5.59 44.07,5.59 v46.99,8.51
BOOT0  (via drill 0.25 pad 0.51)
  Top 0.152: v41.27,6.6 46.23,6.6 49.78,3.05 J2.6 | R4.1 28.45,6.22 28.07,6.6 v28.07,6.73 28.42,7.08 U2.60 | SW1.2 25.88,3.45 v25.15,4.19
  Bottom 0.152: v41.27,6.6 41.15,6.73 v28.07,6.73 28.07,5.33 26.8,4.06 25.27,4.06 v25.15,4.19
BOOT1  (via drill 0.25 pad 0.51)
  Top 0.152: U2.28 24.92,19.15 25.4,18.67 v25.91,18.67 | R27.1 R24.2 34.86,17.59 35.2,17.93 v35.2,18.29
  PWR 0.152: v25.91,18.67 26.92,17.65 34.57,17.65 v35.2,18.29 37.72,18.29 42.29,13.72 42.29,8.76 44.58,6.48 47.12,6.48 J2.7
FT_3V3_O  (via drill 0.25 pad 0.51)
  Top 0.305: U5.1 9.42,13.42 R28.1 v8.51,13.02 C36.2 | U5.8 13.68,9.82 v14.1,9.4 C34.2
  PWR 0.305: v14.1,9.4 14.1,9.91 13.46,10.54 8.13,10.54 7.75,10.92 7.75,12.26 v8.51,13.02
GND  (via drill 0.25 pad 0.51, 0.64 pad 1.27)
  Top 0.152: U1.13 45.04,9.74 44.83,9.53 v44.7,9.53
  Top 0.203: C1.2 50.86,18.22 50.8,18.29 | U2.47 20.27,10.72 19.24,11.75 C19.2 | R15.1 36.77,15.49 C23.2 v37.59,15.56
  Top 0.229: v50.93,14.22 50.78,14.08 U1.33 48.78,14.08 v48.51,14.35 48.64,14.48 U1.34 50.67,14.48 v50.93,14.22 | C10.1 46.1,18.16 46.93,18.99 C6.2 | U1.13 45.04,10.88 v45.97,11.81 | v50.93,14.22 52.07,14.22 v52.2,14.35 52.2,15.24 | 52.2,15.24 51.69,15.75 | 52.2,15.24 v52.2,15.88 51.94,16.13 51.44,16.13 | 51.44,16.13 v50.93,16.64 | C4.1 51.5,17.72 50.93,17.14 | 51.12,16 51.24,16.13 51.44,16.13 | C8.2 51.75,15.81 51.94,16
  Top 0.254: U2.31 23.42,20.52 v23.3,20.64 C26.1 | U2.63 29.92,9.92 v29.97,9.97 | C12.1 42.8,18.16 42.04,18.92 v42.04,19.18
  Top 0.279: U2.18 29.92,18.98 v29.97,18.92
  Top 0.305: U5.3 12.39,12.12 v12.7,12.43 | U5.13 13.68,13.41 v13.21,12.94
  Top 0.406: OTG.5 5.43,17.2 v5.66,16.97
  Top 0.508: v12.7,12.43 U5.T
  Top 0.61: C26.1 22.23,21.59 21.84,21.97 | D6.2 14.1,6.86 C34.1 14.59,7.32 | U3.1 14.59,7.32 | 14.59,7.32 14.59,6.51 v14.55,6.48
  other vias: 8.26,17.02 10.79,19.49 28.52,4.65 34.29,10.79 10.16,14.59 12.19,12.94 47.24,13.08 48.51,13.08 45.97,13.08 47.24,11.81 48.51,11.81 47.24,14.35 45.97,14.35 47.5,17.27 46.99,19.81 51.94,18.41 51.94,19.68 52.96,20.45 53.72,19.56 51.94,8.51 52.96,8.51 44.7,8.89 0.64,13.32 0.64,12.31 0.64,11.29 0.64,10.15 7.62,4.45 14,1.5 12,1.5 7.25,14.49 52.7,6.35 51.44,5.08 14.22,19.16 1.98,19.7 1.98,17.28 49.53,25.4 47.62,24.13 50.16,6.35 53.72,18.54 53.72,17.02 53.72,15.88 53.72,14.61 53.72,13.34 53.72,12.06 53.72,10.79 53.72,9.53 51.94,20.45 51.44,6.35 52.7,5.08 47.62,22.86 49.53,22.86 47.62,25.4 49.53,24.13 34.29,10.16 38.1,8.89 40.26,8.89 40.26,10.16 40.26,11.43 34.29,11.43 7.62,3.17 7.62,1.91 20.95,1.91 22.23,1.91 9.14,4.95 10.03,4.95 10.03,4.19 9.14,4.19 16,4.95 16.89,4.95 16.89,4.19 16,4.19 44.07,9.53 44.07,8.89 6.35,14.72 8,15.23 11.81,20.51 13.21,19.49 17.65,20.26 18.41,19.75 42.7,16.37 13.34,17.64 12.06,17.64 12.06,19.49 20.32,9.4 19.3,3.81 15.88,6.48 31.11,10.79 42.06,15.86 46.99,20.7 45.09,20.7 43.81,20.7 10.79,17.64 20.32,8.51 18.03,12.06 31.11,9.53 31.5,8.26 34.29,7.87 34.29,7.24 24.77,1.91 24.13,3.17 18.54,2.54 24.77,9.51 28.32,13.96 28.57,16.12 22.86,22.85 23.5,22.85 25.78,23.1 34.92,14.59 36.2,14.59 37.47,14.59 38.1,17.13 38.48,16.43 38.48,15.54 51.05,11.56 51.05,10.29 14.55,7.05 17.14,16.69 13.97,16.76 8.26,19.88 9.53,19.88 9.53,17.08 9.53,15.24 11.18,7.24 26.92,10.92 38.1,7.24 20.32,4.45 38.48,14.59 21.34,4.45 19.05,16.69 51.5,25.46 51.44,24.13 51.44,22.86 8.26,23.05 9.53,23.05 35.18,6.1 30.11,4.71 7.25,12.71 7.62,24.19 24.13,5.08 32.38,4.45 33.66,4.45 48.9,6.35 34.53,18.3 38.48,19.35 39.88,20.37 39.88,19.04 39.88,17.89 23.75,10.15 24.77,10.15 17.4,14.35 14.61,15.11 25.4,12.32 26.67,12.32 23.5,12.32 17.27,11.68 17.4,10.16 17.4,9.53 29.84,1.91 50.16,5.08 15.24,15.11 22.35,22.34 59.05,19.68 57.78,19.68 55.88,19.68 53.98,20.95 55.88,22.23 57.78,22.23 59.05,22.23 51.37,28 49.47,28 47.56,28 39.5,13.21 39.75,7.62
  pour Top (isolate 0.203, rank 6): -0.64,30.48 60.33,30.48 60.33,18.41 55.12,18.41 55.12,-0.64 -0.64,-0.64
  pour Bottom (isolate 0.203, rank 6): -0.64,30.48 60.33,30.48 60.33,18.41 55.12,18.41 55.12,-0.64 2.54,-0.64 2.54,-2.54 -0.64,-2.54
  pour GND (isolate 0.203, rank 6): -0.64,-1.27 -0.64,30.48 60.33,30.48 60.33,18.41 55.12,18.41 55.12,-0.64 1.27,-0.64 1.27,-1.27
  pour Bottom (isolate 0.254, rank 6, no thermals): 8.26,5.71 17.78,5.71 17.78,0 8.26,0
  pour Top (isolate 0.254, rank 6, no thermals): 8.26,5.71 17.78,5.71 17.78,2.54 30.48,2.54 30.48,-0.25 8.26,-0.25
  pour Bottom (isolate 0.254, rank 6, no thermals): 0,13.97 0,23.5 5.71,23.5 5.71,13.97
  pour Top (isolate 0.254, rank 6, no thermals): 0,13.97 0,23.5 5.71,23.5 5.71,13.97
N$1
  Top 0.229: C5.2 L1.2 58.64,17.72 ANT1.ANT
N$2
  Top 0.203: U1.38 49.04,17.19 | C2.2 48.96,18.1 48.64,18.41 X1.3
  Top 0.229: 49.04,17.19 C2.2
N$3
  Top 0.229: U1.29 51.4,12.48 51.94,11.94 C7.1
N$4
  Top 0.152: U1.39 48.64,16.51 48.51,16.64 47.24,16.64 46.99,16.89 C6.1
N$5
  Top 0.203: U1.37 49.44,16.74 C1.1 49.97,17.34 49.78,17.53 49.78,19.3 X1.1
N$6
  Top 0.229: U1.2 42.9,14.88 L4.1
N$7
  Top 0.406: L4.2 41.27,16.19 L5.1
N$8
  Top 0.229: C3.2 L1.1 C4.2
N$9
  Top 0.279: U2.30 23.92,21.55 C26.2
N$10
  Top 0.152: R6.2 40.01,5.21 40.89,4.32 40.89,2.54 J2.3
N$11  (via drill 0.25 pad 0.51)
  Top 0.152: OTG.4 5.9,17.85 6.48,17.27 v6.48,16 6.54,16.07 D4.1 8.38,16.07 R32.1
  Bottom 0.152: v6.48,16 TP4.T
N$12
  Top 0.152: U2.6 35.03,12.72 C21.1 35.56,12.57 X4.1
N$13
  Top 0.152: U2.5 34.52,12.22 C20.2 37.34,11.56 X4.3
N$14  (via drill 0.25 pad 0.51)
  Top 0.152: R30.1 D2.1 7.08,19.15 6.73,19.15 6.5,19.15 | OTG.2 6.2,19.15 | 6.2,19.15 6.35,19.15 | 6.35,19.15 6.5,19.15 | v6.35,19.43 6.35,19.3 | 6.35,19.3 6.35,19.15 | 6.2,19.15 6.35,19.3 | 6.5,19.15 6.35,19.3
  Bottom 0.152: TP2.T v6.35,19.43
N$15  (via drill 0.25 pad 0.51)
  Top 0.152: R31.1 D3.1 6.71,18.5 6.56,18.5 | OTG.3 6.14,18.5 | 6.14,18.5 6.35,18.5 | 6.35,18.5 6.56,18.5 | v6.35,18.29 6.35,18.5 | 6.14,18.5 v6.35,18.29 | 6.56,18.5 v6.35,18.29
  Bottom 0.152: TP3.T v6.35,18.29
N$17  (via drill 0.25 pad 0.51)
  Top 0.203: 11.7,5.06 11.68,5.08 11.56,5.08
  Top 0.356: USB.1 11.7,5.06 11.56,5.21 11.3,5.46
  Top 0.406: 10.67,5.97 11.3,5.97 11.7,5.57 USB.1 | 11.18,5.46 10.67,5.46 10.03,6.1
  Top 0.61: 11.56,5.21 11.56,5.08 11.18,5.46 10.67,5.97 10.54,6.1 | 10.54,6.1 10.16,6.48 D8.1 8.76,6.6 F2.1 | 10.54,6.1 10.03,6.1 v9.27,6.1 8.64,6.1 8.51,6.1 8.13,6.48
  Bottom 0.203: TP5.T v9.27,6.1
N$18
  Top 0.305: R8.1 C17.1 33.21,8.83 32.47,9.57 U2.1
N$19  (via drill 0.25 pad 0.51)
  Top 0.152: U2.20 28.92,20.28 29.21,20.57 30.86,20.57 31.24,20.19 v31.24,19.94 | v35.43,20.32 35.75,20.32 R18.2
  PWR 0.152: v35.43,20.32 31.62,20.32 v31.24,19.94
N$20  (via drill 0.25 pad 0.51)
  Top 0.152: U2.21 28.42,20.55 28.77,20.89 31.05,20.89 32,19.94 v32,19.81 | v35.43,19.3 35.75,19.3 R19.2
  PWR 0.152: v35.43,19.3 32.51,19.3 v32,19.81
N$21  (via drill 0.25 pad 0.51)
  Top 0.152: U2.22 27.92,20.81 28.32,21.21 31.62,21.21 v32,20.83 | v35.43,21.34 35.75,21.34 R20.2
  PWR 0.152: v35.43,21.34 32.51,21.34 v32,20.83
N$22  (via drill 0.25 pad 0.51)
  Top 0.152: U2.23 27.42,20.82 28.13,21.53 31.94,21.53 v32,21.59 | v35.43,22.35 35.75,22.35 R21.2
  PWR 0.152: v35.43,22.35 35.31,22.48 32.89,22.48 v32,21.59
N$23
  Top 0.152: U2.26 25.92,20.84 27.94,22.86 31.75,22.86 32.51,22.1 32.51,21.02 R22.2
N$24
  Top 0.152: U2.27 25.42,20.85 27.81,23.24 31.88,23.24 32.89,22.23 32.89,21.65 R23.2
N$25
  Top 0.152: SW1.1 29.23,5.04 R25.1
N$26
  Top 0.152: 33.97,15.49 C24.2
  Top 0.203: R15.2 33.97,15.49 | U2.12 33.75,15.72 C24.2
N$27
  Top 0.152: 33.97,16.51 C24.1
  Top 0.203: R17.2 33.97,16.51 | U2.13 33.68,16.22 C24.1
N$28  (via drill 0.25 pad 0.51)
  Top 0.152: R3.2 v48.07,8.51
  Bottom 0.152: BLE_SWD.4 44.7,4.83 48.07,8.19 v48.07,8.51
N$29
  Top 0.152: R7.2 33.27,6.22 33.91,5.59 42.29,5.59 43.56,4.32 43.56,2.41 J2.4
N$30  (via drill 0.25 pad 0.51)
  Top 0.203: U5.7 13.03,9.96 v13.08,9.91 | R35.2 v12.06,9.27
  PWR 0.203: v12.06,9.27 12.45,9.27 v13.08,9.91
N$31
  Top 0.152: USR1.+ R9.2
N$32
  Top 0.203: U5.6 12.38,9.85 13.08,9.14 R36.2
N$33  (via drill 0.25 pad 0.51)
  Top 0.152: U5.15 12.38,15.17 v12.45,15.24 | R33.1 25.4,6.6 v25.27,6.73
  Bottom 0.152: v12.45,15.24 12.95,15.75 17.91,15.75 21.72,11.94 21.72,10.29 v25.27,6.73
N$34  (via drill 0.25 pad 0.51)
  Top 0.152: U5.2 10.36,12.77 10.16,12.57 v10.16,9.65 | R34.1 26.35,6.16 26.04,6.48 v26.04,6.73
  PWR 0.152: v26.04,6.73 25.53,7.24 20,7.24 18.54,8.7 10.73,8.7 10.16,9.27 v10.16,9.65
N$35
  Top 0.152: USR2.+ R10.2
N$36
  Top 0.152: BT.+ R14.2
N$37
  Top 0.152: U2.56 26.42,7.11 27.24,6.29 27.24,6.16 R5.1
N$38  (via drill 0.25 pad 0.51)
  Top 0.152: U5.9 14.82,11.47 14.99,11.3 v14.99,10.41 | R28.2 9.34,12.13 v9.53,12.32
  Bottom 0.152: v14.99,10.41 14.61,10.79 11.05,10.79 v9.53,12.32
N$39  (via drill 0.25 pad 0.51)
  Top 0.406: OTG.1 5.3,19.8 5.41,19.91 | v6.35,21.84 7.37,21.84 7.49,21.72
  Top 0.61: 5.41,19.91 5.44,19.91 7.11,21.59 F1.1 7.49,21.72 7.49,22.8 D7.1
  Bottom 0.406: TP1.T v6.35,21.84
  pour Top (no thermals): 4.32,19.94 4.7,19.94 5.71,20.95 5.71,23.11 6.1,23.5 7.87,23.5 8.13,23.24 8.13,20.57 8,20.45 6.99,20.45 6.1,19.56 4.32,19.56 4.19,19.68 4.19,19.81
N$40  (via drill 0.25 pad 0.51)
  Top 0.152: R2.2 v50.86,8.51
  Bottom 0.152: v50.86,8.51 50.35,9.02 47.75,9.02 47.5,8.76 47.5,8.13 43.18,3.81 BLE_SWD.3
N$41  (via drill 0.25 pad 0.51)
  Top 0.152: U5.11 15.12,12.77 v15.18,12.83 | v0.64,9.14 RX.-
  Bottom 0.152: v15.18,12.83 15.24,12.83 15.49,12.57 15.49,10.16 15.24,9.91 14.35,9.91 13.84,10.41 1.91,10.41 v0.64,9.14
N$42
  Top 0.152: PWR.+ R16.2
N$43  (via drill 0.25 pad 0.51)
  Top 0.152: U5.5 11.72,10.07 v10.92,9.27 | v0.64,8.13 TX.-
  Bottom 0.152: v0.64,8.13 1.65,9.14 10.79,9.14 v10.92,9.27
N$44
  Top 0.152: RX.+ R37.1
N$45
  Top 0.152: TX.+ R38.1
N$46  (via drill 0.25 pad 0.51)
  Top 0.152: 12.35,5.94 v12.19,6.1
  Top 0.203: R35.1 D5.1 12.35,6.45 12.35,6.1 | 12.35,6.1 USB.2 | v12.19,6.1 12.35,6.1
  Bottom 0.152: v12.19,6.1 TP6.T
N$47  (via drill 0.25 pad 0.51)
  Top 0.152: v13.21,6.1 13,6.1 | 13,6.29 13.01,6.29 v13.21,6.1 | 13,5.89 13.01,5.89 v13.21,6.1
  Top 0.203: R36.1 D6.1 13,6.65 13,6.29 13,6.1 13,5.89 USB.3
  Bottom 0.152: TP7.T v13.21,6.1
OTG_FS_DM
  Top 0.152: R30.2 9.59,18.61 14.41,18.61 19.05,13.97 19.05,13.21 20.04,12.22 U2.44
OTG_FS_DP
  Top 0.152: R31.2 9.53,18.29 14.22,18.29 18.67,13.84 18.67,13.08 20.03,11.72 U2.45
OTG_FS_SOF
  Top 0.152: U2.41 20.32,13.72 20.07,13.97 20.07,17.72 R13.1
PA0/UART2_CTS  (via drill 0.25 pad 0.51)
  Top 0.152: U2.14 22.65,16.72 v22.61,16.76
  Bottom 0.152: J1.1 10,24.16 16.89,17.27 22.1,17.27 v22.61,16.76
PA1/UART2_RTS  (via drill 0.25 pad 0.51)
  Top 0.152: U2.15 24.05,17.22 v24,17.27
  Bottom 0.152: J1.7 17.62,23.4 20.83,20.19 22.35,20.19 24,18.54 v24,17.27
PA2/UART2_TX  (via drill 0.25 pad 0.51)
  Top 0.152: v20.7,18.54 21.84,18.54 22.1,18.29 24.89,18.29 25.4,17.78 U2.16
  Bottom 0.152: v20.7,18.54 20.57,18.41 17.91,18.41 12.54,23.78 J1.3
PA3/UART2_RX  (via drill 0.25 pad 0.51)
  Top 0.152: U2.17 30.52,19.81 30.52,18.58 30.1,18.16 25.46,18.16 24.96,18.67 22.61,18.67 v22.48,18.8
  Bottom 0.152: J1.5 15.08,23.91 19.56,19.43 21.84,19.43 v22.48,18.8
PA15  (via drill 0.25 pad 0.51)
  Top 0.152: U2.50 23.42,5.77 v23.37,5.71 | R10.1 4.83,13.34 6.99,11.18 v6.99,6.99
  PWR 0.152: v23.37,5.71 20.19,5.71 18.16,7.75 7.75,7.75 v6.99,6.99
PB3/PWM0/I2C2_SDA/SWO  (via drill 0.25 pad 0.51)
  Top 0.152: U2.55 25.92,10.93 v26.42,11.43
  Bottom 0.152: J1.25 40.48,23.34 35.94,18.8 34.16,18.8 31.24,15.88 31.24,12.19 30.48,11.43 v26.42,11.43
PB5  (via drill 0.25 pad 0.51)
  Top 0.152: R14.1 5.21,11.3 5.71,10.79 v5.71,6.99 | U2.57 26.92,7.37 27.3,6.99 v27.43,6.99
  PWR 0.152: v27.43,6.99 26.67,6.22 25.02,6.22 24.38,6.86 19.94,6.86 18.41,8.38 6.35,8.38 5.71,7.75 v5.71,6.99
PB6/I2C1_SCL/UART1_TX  (via drill 0.25 pad 0.51)
  Top 0.152: U2.58 27.42,12.69 v27.43,12.7
  Bottom 0.152: J1.21 35.02,24.73 32.51,22.23 32.51,19.18 27.43,14.1 v27.43,12.7
PB7/I2C1_SDA/UART1_RX  (via drill 0.25 pad 0.51)
  Top 0.152: U2.59 27.92,12.3 28.45,12.83 29.21,12.83 v29.72,12.32
  Bottom 0.152: J1.23 36.45,23.24 34.54,23.24 33.27,21.97 33.27,18.92 29.72,15.37 v29.72,12.32
PB8/I2C1_SCL  (via drill 0.25 pad 0.51)
  Top 0.152: U2.61 28.92,12.28 v28.96,12.32
  Bottom 0.152: J1.22 36.58,26.09 36.58,24.26 35.94,23.62 34.42,23.62 32.89,22.1 32.89,19.05 28.96,15.11 v28.96,12.32
PB9/I2C1_SDA  (via drill 0.25 pad 0.51)
  Top 0.152: U2.62 29.42,11.13 v30.61,12.32
  Bottom 0.152: v30.61,12.32 30.61,15.75 33.66,18.8 33.66,21.84 34.67,22.86 37.59,22.86 39.12,24.38 39.12,26.09 J1.24
PB10/PWM1/I2C2_SCL
  Top 0.152: U2.29 24.42,20.86 26.67,23.11 26.67,25.53 27.05,25.91 41.84,25.91 J1.27
PB12/SPI2_SS  (via drill 0.25 pad 0.51)
  Top 0.152: U2.33 21.34,17.78 v21.59,18.03
  Bottom 0.152: J1.2 11.3,25.97 11.3,23.37 16.76,17.91 21.46,17.91 v21.59,18.03
PB13/SPI2_SCK  (via drill 0.25 pad 0.51)
  Top 0.152: U2.34 21.54,17.22 22.1,17.78 v24.51,17.78
  Bottom 0.152: v24.51,17.78 24.51,18.54 22.48,20.57 20.95,20.57 18.92,22.61 18.92,25.97 J1.8
PB14/SPI2_MISO  (via drill 0.25 pad 0.51)
  Top 0.152: U2.35 21.95,16.72 22.42,16.26 23.11,16.26 v23.75,15.62
  Bottom 0.152: J1.6 16.38,25.97 16.38,23.11 19.68,19.81 22.23,19.81 23.5,18.54 23.5,15.88 v23.75,15.62
PB15/SPI2_MOSI  (via drill 0.25 pad 0.51)
  Top 0.152: U2.36 21.88,16.22 22.48,15.62 v22.86,15.62
  Bottom 0.152: v22.86,15.62 23.11,15.88 23.11,17.4 21.46,19.05 17.78,19.05 13.84,22.99 13.84,25.97 J1.4
PC0/ADC_IN10  (via drill 0.25 pad 0.51)
  Top 0.152: U2.8 33.52,13.72 v33.66,13.59
  Bottom 0.152: J1.26 41.66,26.09 41.66,24 33.66,16 v33.66,13.59
PC1/ADC_IN11  (via drill 0.25 pad 0.51)
  Top 0.152: U2.9 34.04,14.22 v34.16,14.1
  Bottom 0.152: J1.28 44.2,26.09 44.2,24.26 43.43,23.5 41.66,23.5 34.04,15.88 34.04,14.22 v34.16,14.1
PC2/ADC_IN12  (via drill 0.25 pad 0.51)
  Top 0.152: U2.10 25.67,14.72 v24.77,15.62
  Bottom 0.152: J1.13 25.24,16.1 v24.77,15.62
PC3/ADC_IN13  (via drill 0.25 pad 0.51)
  Top 0.152: U2.11 26.44,15.22 v26.04,15.62
  Bottom 0.152: J1.14 26.42,26.09 26.42,16 v26.04,15.62
PC4/ADC1_IN14  (via drill 0.25 pad 0.51)
  Top 0.152: U2.24 26.92,20.82 28.13,22.04 v28.57,22.04
  Bottom 0.152: J1.15 27.78,22.83 v28.57,22.04
PC5/ADC1_IN15  (via drill 0.25 pad 0.51)
  Top 0.152: U2.25 26.42,20.83 28.13,22.54 28.89,22.54 v29.34,22.1
  Bottom 0.152: J1.16 29.08,25.97 29.08,22.35 v29.34,22.1
PC6/UART6_TX  (via drill 0.25 pad 0.51)
  Top 0.152: U2.37 21.87,15.72 22.48,15.11 v24.26,15.11
  Bottom 0.152: J1.17 30.32,22.32 26.8,18.8 26.8,15.49 26.42,15.11 v24.26,15.11
PC7/UART6_RX  (via drill 0.25 pad 0.51)
  Top 0.152: U2.38 21.86,15.22 22.48,14.61 v24.77,14.61
  Bottom 0.152: v24.77,14.61 26.42,14.61 27.18,15.37 27.18,18.67 31.5,22.99 31.5,26.09 J1.18
PC8  (via drill 0.25 pad 0.51)
  Top 0.152: U2.39 21.86,14.72 22.61,13.97 v24.26,13.97
  Bottom 0.152: J1.19 32.86,23.72 27.56,18.41 27.56,15.24 26.29,13.97 v24.26,13.97
PC9  (via drill 0.25 pad 0.51)
  Top 0.152: U2.40 21.72,14.22 22.61,13.34 v24.77,13.34
  Bottom 0.152: J1.20 34.04,26.09 34.04,24.38 27.94,18.29 27.94,15.11 26.16,13.34 v24.77,13.34
PD2  (via drill 0.25 pad 0.51)
  Top 0.152: R9.1 5,12.32 6.35,10.97 v6.35,7.62 | U2.54 25.42,7.58 24.19,6.35 v24.11,6.35
  PWR 0.152: v24.11,6.35 20,6.35 18.29,8.06 6.79,8.06 v6.35,7.62
RST_!BTN  (via drill 0.25 pad 0.51)
  Top 0.152: v23.11,5.08 22.38,5.08 D1.-
  Top 0.203: D1.- 22.29,4.38 23.27,3.4 RST.1
  PWR 0.152: v42.55,6.1 44.58,6.1 45.97,4.7 45.97,2.54 J2.5
  Bottom 0.152: J1.29 45.56,24.48 41.53,20.45 41.53,14.48 42.04,13.97 42.04,6.22 | 41.91,6.1 36.32,6.1 33.91,3.68 24.51,3.68 v23.11,5.08 | 41.91,6.1 42.04,6.1 | 42.04,6.1 42.16,6.1 | 42.16,6.1 v42.55,6.1 | 42.04,6.22 42.04,6.1 | 41.91,6.1 42.04,6.22 | 42.04,6.22 42.16,6.1
ST_!RESET
  Top 0.152: U2.7 25.54,13.22 21.27,8.95 C22.2 | C22.2 R11.2 | C22.2 22,6.48 D1.+
ST_SWCLK  (via drill 0.25 pad 0.51)
  Top 0.152: R6.1 32.26,5.21 31.81,4.76 v31.5,4.76 | U2.49 22.86,8.38 v22.48,8.76
  PWR 0.152: v31.5,4.76 31.3,4.76 27.3,8.76 v22.48,8.76
ST_SWDIO  (via drill 0.25 pad 0.51)
  Top 0.152: R7.1 32,6.22 31.5,5.71 v31.5,5.46 | U2.46 22.75,11.22 v22.99,11.46
  PWR 0.152: v31.5,5.46 31.11,5.46 25.46,11.11 25.38,11.2 25.12,11.46 v22.99,11.46
USART1_RX/OTG_FS_ID  (via drill 0.25 pad 0.51)
  Top 0.152: R32.2 v10.03,16.13 | U2.43 21.7,12.72 v21.72,12.7 | v25.65,4.7 25.65,5.02 R33.2
  PWR 0.152: UART.1 29.46,3.81 26.54,3.81 v25.65,4.7
  Bottom 0.152: v10.03,16.13 18.29,16.13 v21.72,12.7 22.1,12.32 22.1,10.41 25.15,7.37 26.16,7.37 26.54,6.99 26.54,6.22 25.65,5.33 v25.65,4.7
USART1_TX/OTG_FS_VBUS  (via drill 0.25 pad 0.51)
  Top 0.152: R12.1 19.68,17.02 19.68,13.84 20.31,13.22 U2.42 21.96,13.22 v22.48,12.7 | R34.2 v26.42,4.7
  PWR 0.152: v26.42,4.7 26.92,4.19 31.62,4.19 UART.2
  Bottom 0.152: v26.42,4.7 26.42,5.59 26.92,6.1 26.92,7.11 26.29,7.75 25.27,7.75 22.48,10.54 v22.48,12.7
USB5V  (via drill 0.25 pad 0.51)
  Top 0.305: U5.10 15.31,12.12 | R12.2 16.7,17.59 15.11,19.18 v15.11,20.45
  Top 0.61: C33.1 16.26,12.32 | 16.26,12.32 15.88,12.32 | 15.88,12.32 15.68,12.12 15.31,12.12 | C28.2 16,9.7 U3.3 | C28.2 v16,11.68 | v16,11.68 16,12 C33.1 | v16,11.68 15.62,12.06 | F1.2 10.73,22.04 C32.1 13.14,22.04 C30.2 13.93,21.97 U4.3 15.11,20.78 v15.11,20.45 | v8.51,11.18 F2.2 9.02,10.16 v9.02,11.18 v8.51,11.18 | C37.1 16.19,12.38 16.26,12.32 | 15.88,12.32 16.13,12.57 | v8.51,11.18 8.26,11.18 8,10.92 8,9.91 | C28.2 16,11.18 v16.51,11.68 16.32,11.87 C33.1
  PWR 0.61: v8.51,11.18 8.64,11.3 | v16.51,11.68 v16,11.68 | 16.13,19.43 v15.11,20.45 v15.49,20.07 15.49,20.45 16.26,21.21
  PWR 0.813: 8.64,11.3 15.62,11.3 v16,11.68 16.26,11.94 16.26,19.43 16.26,20.45 | 16.26,20.45 15.49,20.45 v15.11,20.45 | J1.11 22.7,24.22 20.32,21.84 17.02,21.84 16.45,21.27 16.26,21.08 | 16.26,21.08 16,20.83 | 16.26,20.45 16.26,21.08
  Bottom 0.508: v16.51,11.68 v16,11.68 | v15.49,20.07 v15.11,20.45
  Bottom 0.61: v9.02,11.18 v8.51,11.18
  pour Top (isolate 0.254, no thermals): 10.79,20.7 9.78,20.7 9.65,20.83 9.65,22.48 10.03,22.86 14.86,22.86 15.49,22.23 15.75,21.97 15.75,20.07 15.49,19.81 14.35,19.81 13.97,20.19 13.97,20.95 13.72,21.21 11.3,21.21
VCC  (via drill 0.25 pad 0.51)
  Top 0.203: R17.1 36.77,16.51 C23.1 v37.59,16.45 | R11.1 19.68,5.46 v19.3,5.08
  Top 0.229: U1.1 44.28,15.28 | 44.28,15.28 44.07,15.49 | 44.07,15.62 44.09,15.62 44.42,15.29 44.29,15.29 44.28,15.28 | U1.12 43.65,10.88 43.56,10.79
  Top 0.279: U2.19 29.42,19.01 v29.21,18.8
  Top 0.406: U2.32 22.86,20.07 22.73,20.19 | R38.2 R37.2 v4.25,9.65 R16.1 | U2.48 20.07,10.16 v19.43,10.79 | R25.2 C15.1 30.48,7.24 v30.54,7.3 | U2.64 30.48,7.37 v30.54,7.3 | R8.2 30.61,7.24 v30.54,7.3
  Top 0.508: C19.1 19.37,10.86 v19.43,10.79
  Top 0.61: 22.73,20.19 22.48,20.45 21.97,20.45 21.4,21.02 C27.2 R26.1 v19.81,20.45 | 44.07,15.49 43.94,15.62 v43.94,16.38 43.94,17.08 C13.2 | v42.8,11.68 C14.2 43.56,10.79 | R1.2 v45.47,9.02 | U3.2 18.2,7.32 C35.+ 18.54,6.48 C29.2 v19.3,5.08 | v31.62,19.05 C25.2 33.47,18.35 33.97,17.84 R24.1 | R13.2 17.4,18.67 v17.14,18.41
  Bottom 0.508: v19.81,5.08 v19.3,5.08
  Bottom 0.61: v19.3,5.08 19.3,10.67 v19.43,10.79
  other vias: 19.3,5.59
  pour PWR (isolate 0.203, rank 6, no thermals): -0.64,-1.91 -0.64,30.48 60.33,30.48 60.33,18.41 55.12,18.41 55.12,-0.64 1.91,-0.64 1.91,-1.91
  pour Top (isolate 0.254, no thermals): 20.7,5.08 20.7,5.71 arc90 20.57,5.84 20.07,5.84 19.81,6.1 19.81,7.62 19.43,8 16.89,8 16.64,7.75 16.64,5.97 18.03,4.57 20.19,4.57
VCC2  (via drill 0.25 pad 0.51)
  Top 0.406: 21.46,26.04 21.46,26.03 | 21.46,26.03 21.46,24.13 20.19,22.86 20.07,22.73 | R26.2 v19.81,22.73 20.07,22.73 | R26.2 18.48,21.91 C31.2 | 21.46,26.03 J1.12 | R26.2 19.81,22.48 20.07,22.73
  Top 0.61: U4.2 18.23,22.16 C31.2
  Bottom 0.406: v19.81,22.73 20.07,22.73 21.46,24.13 21.46,26.04 22.23,26.8 | 22.23,26.8 22.35,26.92 | 22.23,26.8 J1.12
  pour Top (isolate 0.254, no thermals): 16.38,23.24 19.94,23.24 20.19,22.99 20.19,21.72 20.07,21.59 16.26,21.59 16.13,21.72 16.13,22.99
VDD_PA
  Top 0.229: U1.30 51.76,12.88 52.32,12.32 52.32,11.3 52.58,11.05 L3.1 C9.2
XL1_32768I
  Top 0.229: U1.46 45.84,16.64 44.96,17.53 44.64,17.53 C12.2 44.01,18.22 42.93,19.3 X2.1
XL1_32768I1
  Top 0.152: X3.1 36.7,9.27 36.2,8.76 C18.2 34.61,8.76 33.72,9.65 33.72,11.05 33.05,11.72 U2.4
XL2_32768E
  Top 0.229: U1.45 46.24,16.88 45.02,18.1 C10.2 45.02,18.22 45.97,19.18 X2.2
XL2_32768E1
  Top 0.152: X3.2 36.7,7.24 36.2,7.75 C16.2 33.4,9.53 33.4,10.92 33.1,11.22 U2.3
(copper drawn outside any net)
  shapes: Top area x1

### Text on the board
Top: L1
GND: L2
PWR: L3
Bottom: L4
tNames: 2 | 30 | 1 | 29 | BLE | 3V3 | GND | CLK | DIO | RST | RST | BOOT0 | RX1 | TX1 | BOOT0 | BOOT1 | UART | 3V3 | GND | CLK | DIO | RST | ST
bNames: BLE Carbon | v1.0 by Seeed & 96Boards | 08/19/2016 | 3V3 | GND | CLK | DIO | RST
